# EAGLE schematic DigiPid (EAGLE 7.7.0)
DESIGNER: A. Stummer; GROUP: J. Thywissen Labs; RELEASE_DATE: 2016 Sept; REV: A; TITLE: DigiPid - Digital PID

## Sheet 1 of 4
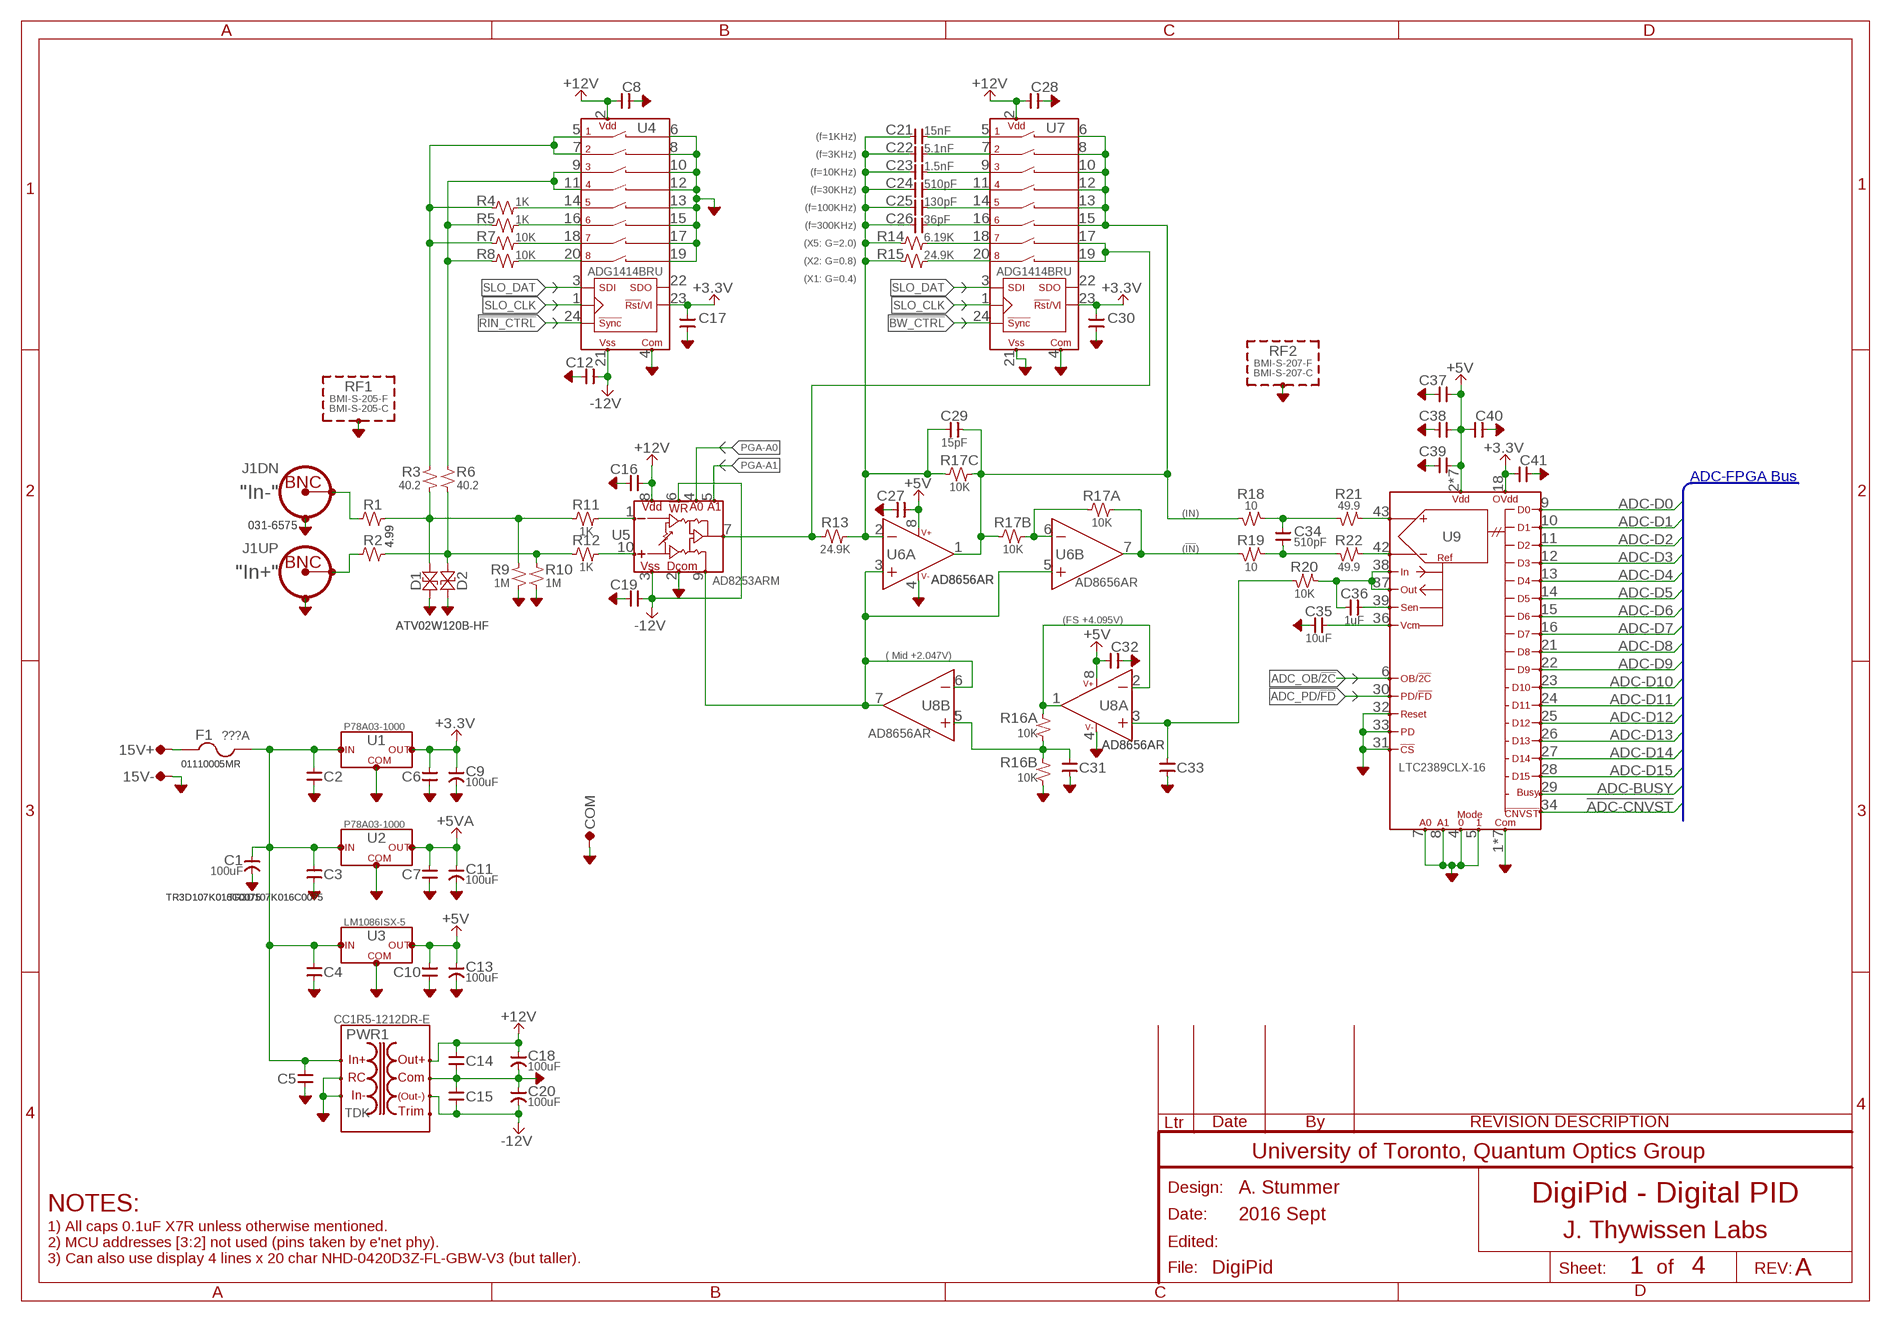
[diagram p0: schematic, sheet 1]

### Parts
15V+  TP-1.5MM  [TP,1.5MM]
15V-  TP-1.5MM  [TP,1.5MM]
C1  100uF  CAP-POL--EIA7343  [7343]
C2  0.1uF  CAP-H-0805  [2012(0805)]
C3  0.1uF  CAP-H-0805  [2012(0805)]
C4  0.1uF  CAP-H-0805  [2012(0805)]
C5  0.1uF  CAP-H-0805  [2012(0805)]
C6  0.1uF  CAP-H-0805  [2012(0805)]
C7  0.1uF  CAP-H-0805  [2012(0805)]
C8  0.1uF  CAP-H-0805  [2012(0805)]
C9  100uF  CAP-POL--EIA7343  [7343]
C10  0.1uF  CAP-H-0805  [2012(0805)]
C11  100uF  CAP-POL--EIA7343  [7343]
C12  0.1uF  CAP-H-0805  [2012(0805)]
C13  100uF  CAP-POL--EIA7343  [7343]
C14  0.1uF  CAP-H-0805  [2012(0805)]
C15  0.1uF  CAP-H-0805  [2012(0805)]
C16  0.1uF  CAP-H-0805  [2012(0805)]
C17  0.1uF  CAP-V-0805  [2012(0805)]
C18  100uF  CAP-POL--EIA7343  [7343]
C19  0.1uF  CAP-H-0805  [2012(0805)]
C20  100uF  CAP-POL--EIA7343  [7343]
C21  15nF  CAP-H-0805  [2012(0805)]
C22  5.1nF  CAP-H-0805  [2012(0805)]
C23  1.5nF  CAP-H-0805  [2012(0805)]
C24  510pF  CAP-H-0805  [2012(0805)]
C25  130pF  CAP-H-0805  [2012(0805)]
C26  36pF  CAP-H-0805  [2012(0805)]
C27  0.1uF  CAP-H-0805  [2012(0805)]
C28  0.1uF  CAP-H-0805  [2012(0805)]
C29  15pF  CAP-H-0805  [2012(0805)]
C30  0.1uF  CAP-V-0805  [2012(0805)]
C31  0.1uF  CAP-H-0805  [2012(0805)]
C32  0.1uF  CAP-H-0805  [2012(0805)]
C33  0.1uF  CAP-H-0805  [2012(0805)]
C34  510pF  CAP-V-0805  [2012(0805)]
C35  10uF  CAP-H-0805  [2012(0805)]
C36  1uF  CAP-H-0805  [2012(0805)]
C37  0.1uF  CAP-H-0805  [2012(0805)]
C38  0.1uF  CAP-H-0805  [2012(0805)]
C39  0.1uF  CAP-H-0805  [2012(0805)]
C40  0.1uF  CAP-H-0805  [2012(0805)]
C41  0.1uF  CAP-H-0805  [2012(0805)]
COM  TP-1MM  [TP-0.042C]
D1  ATV02W120B-HF  TVS,BIPOLAR-SOD123  [SOD123]
D2  ATV02W120B-HF  TVS,BIPOLAR-SOD123  [SOD123]
F1  ???A  FUSE-5X20-4  [FUSE]
J1  031-6575  CONN:BNC,DUAL-BOMAR_364A  [CONN:BNC,DUAL(BOMAR)]
PWR1  CC1R5-1212DR-E  DC-DC:CCP-__-E(TDK1.5-25W)-CC1R5-R-E  [DC-DC:CC1R5-XXXXX-R-E(TDK/LAMBDA)]
R1  4.99  R-H-0805  [2012(0805)]
R2  4.99  R-H-0805  [2012(0805)]
R3  40.2  R-V-0805  [2012(0805)]
R4  1K  R-H-0805  [2012(0805)]
R5  1K  R-H-0805  [2012(0805)]
R6  40.2  R-V-0805  [2012(0805)]
R7  10K  R-H-0805  [2012(0805)]
R8  10K  R-H-0805  [2012(0805)]
R9  1M  R-V-0805  [2012(0805)]
R10  1M  R-V-0805  [2012(0805)]
R11  1K  R-H-0805  [2012(0805)]
R12  1K  R-H-0805  [2012(0805)]
R13  24.9K  R-H-0805  [2012(0805)]
R14  6.19K  R-H-0805  [2012(0805)]
R15  24.9K  R-H-0805  [2012(0805)]
R16  10K  R-4PAK-0603  [PANASONIC_EXB-V8V(QUAD-R-PACK)]
R17  10K  R-4PAK-0603  [PANASONIC_EXB-V8V(QUAD-R-PACK)]
R18  10  R-H-0805  [2012(0805)]
R19  10  R-H-0805  [2012(0805)]
R20  10K  R-H-0805  [2012(0805)]
R21  49.9  R-H-0805  [2012(0805)]
R22  49.9  R-H-0805  [2012(0805)]
RF1  BMI-S-205-F  RF-SHIELD-38X25MM(BMI-S-205-F)  [RF-SHIELD,38X25MM(BMI-S-205-F)]
RF2  BMI-S-207-F  RF-SHIELD-44X44MM(BMI-S-207-F)  [RF-SHIELD,44X44MM(BMI-S-207-F)]
U1  P78A03-1000  REGULATOR:3PIN-SMPS(V-OR-H)  [TO220-SMPS]
U2  P78A03-1000  REGULATOR:3PIN-SMPS(V-OR-H)  [TO220-SMPS]
U3  LM1086ISX-5  REGULATOR:3PIN-TO263  [TO263]
U4  ADG1414BRU  SWITCH,8PST-SERIAL-TSSOP24  [TSSOP-24]
U5  AD8253ARM  ANALOG,INT-AMP-PROG#1-MSOP10  [MSOP10]
U6  AD8656AR  OPAMP:AD8___(DUAL)-SOIC-8  [SOIC-8]
U7  ADG1414BRU  SWITCH,8PST-SERIAL-TSSOP24  [TSSOP-24]
U8  AD8656AR  OPAMP:AD8___(DUAL)-SOIC-8  [SOIC-8]
U9  LTC2389CLX-16  ADC,LTC2389-16-LQFP48  [QFP48]

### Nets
!ADC-CNVST: U9.34(!CNVST) ; also sheet 3
!BW_CTRL: U7.24(!SYNC) ; also sheet 4
!RIN_CTRL: U4.24(!SYNC) ; also sheet 4
+3.3V [Power]: C6.1 C9.+VE(POS) C17.2 C30.2 C41.1 U1.3(OUT) U4.23(!RST!/VL) U7.23(!RST!/VL) U9.18(OVDD) ; also sheet 2,3,4
+5V [Power]: C10.1 C13.+VE(POS) C27.1 C32.1 C37.1 C38.1 C39.1 C40.1 U3.4(OUT) U6.8(PWR:V++) U8.8(PWR:V++) U9.2(VDD) U9.3(VDD) U9.19(VDD) U9.40(VDD) U9.45(VDD) U9.46(VDD) U9.47(VDD) ; also sheet 2,3
+5VA [Power]: C7.1 C11.+VE(POS) U2.3(OUT) ; also sheet 4
+12V [Power]: C8.1 C14.1 C16.1 C18.+VE(POS) C28.1 PWR1.+VOUT(+OUT) U4.2(VDD) U5.8(VDD) U7.2(VDD) ; also sheet 2
-12V [Power]: C12.1 C15.2 C19.1 C20.-VE(NEG) PWR1.-VOUT(-OUT) U4.21(VSS) U5.3(VSS) U5.6(!WR) ; also sheet 2
ADC-BUSY: U9.29(BUSY) ; also sheet 3
ADC-D0: U9.9(D0) ; also sheet 3
ADC-D1: U9.10(D1) ; also sheet 3
ADC-D2: U9.11(D2) ; also sheet 3
ADC-D3: U9.12(D3) ; also sheet 3
ADC-D4: U9.13(D4) ; also sheet 3
ADC-D5: U9.14(D5) ; also sheet 3
ADC-D6: U9.15(D6) ; also sheet 3
ADC-D7: U9.16(D7) ; also sheet 3
ADC-D8: U9.21(D8) ; also sheet 3
ADC-D9: U9.22(D9) ; also sheet 3
ADC-D10: U9.23(D10) ; also sheet 3
ADC-D11: U9.24(D11) ; also sheet 3
ADC-D12: U9.25(D12) ; also sheet 3
ADC-D13: U9.26(D13) ; also sheet 3
ADC-D14: U9.27(D14) ; also sheet 3
ADC-D15: U9.28(D15) ; also sheet 3
ADC_OB/!2C: U9.6(OB!2C) ; also sheet 4
ADC_PD/!FD: U9.30(PD!FD) ; also sheet 4
AGND: 15V-.TP C1.-VE(NEG) C2.2 C3.2 C4.2 C5.2 C6.2 C7.2 C8.2 C9.-VE(NEG) C10.2 C11.-VE(NEG) C12.2 C13.-VE(NEG) C14.2 C15.1 C16.2 C17.1 C18.-VE(NEG) C19.2 C20.+VE(POS) C27.2 C28.2 C30.1 C31.2 C32.2 C33.2 C35.1 C37.2 C38.2 C39.2 C40.2 C41.2 COM.TP D1.C(TOTHER) D2.C(TOTHER) J1.LWR-COM(DN:SHIELD2) J1.UPR-COM(UP:SHIELD2) PWR1.-VIN(-IN) PWR1.COM PWR1.RC R9.1 R10.1 R16.2A RF1.1(SHIELD) RF1.2(SHIELD) RF1.3(SHIELD) RF1.4(SHIELD) RF1.5(SHIELD) RF1.6(SHIELD) RF1.7(SHIELD) RF1.8(SHIELD) RF1.9(SHIELD) RF1.10(SHIELD) RF1.11(SHIELD) RF1.12(SHIELD) RF1.13(SHIELD) RF1.14(SHIELD) RF1.15(SHIELD) RF1.16(SHIELD) RF1.17(SHIELD) RF1.18(SHIELD) RF1.19(SHIELD) RF1.20(SHIELD) RF1.21(SHIELD) RF1.22(SHIELD) RF1.23(SHIELD) RF1.25(SHIELD) RF2.1(SHIELD) RF2.2(SHIELD) RF2.3(SHIELD) RF2.4(SHIELD) RF2.5(SHIELD) RF2.6(SHIELD) RF2.7(SHIELD) RF2.8(SHIELD) RF2.9(SHIELD) RF2.10(SHIELD) RF2.11(SHIELD) RF2.12(SHIELD) RF2.13(SHIELD) RF2.14(SHIELD) RF2.15(SHIELD) RF2.16(SHIELD) RF2.17(SHIELD) RF2.18(SHIELD) RF2.19(SHIELD) RF2.20(SHIELD) RF2.21(SHIELD) RF2.22(SHIELD) RF2.23(SHIELD) RF2.24(SHIELD) RF2.25(SHIELD) RF2.26(SHIELD) RF2.27(SHIELD) RF2.28(SHIELD) RF2.29(SHIELD) RF2.30(SHIELD) RF2.31(SHIELD) RF2.32(SHIELD) U1.2(COM) U2.2(COM) U3.1(COM) U4.4(COM) U4.6(D1) U4.8(D2) U4.10(D3) U4.12(D4) U4.13(D5) U4.15(D6) U4.17(D7) U4.19(D8) U5.2(DGND) U6.4(PWR:V-) U7.4(COM) U7.21(VSS) U8.4(PWR:V-) U9.1(COM) U9.4(MODE0) U9.5(MODE1) U9.7(A0) U9.8(A1) U9.17(COM) U9.20(COM) U9.31(!CS) U9.32(RESET) U9.33(PD) U9.35(COM) U9.41(COM) U9.44(COM) U9.48(COM) ; also sheet 2,3,4
N$1: R3.2 R4.1 R7.1 U4.5(S1) U4.7(S2)
N$2: R5.1 R6.2 R8.1 U4.9(S3) U4.11(S4)
N$3: R13.1 U5.7(OUT) U7.17(D7) U7.19(D8)
N$4: U5.9(REF) U6.3(A:+IN) U6.5(B:+IN) U8.6(B:-IN) U8.7(B:OUT)
N$5: R22.1 U9.42(IN-)
N$6: R21.1 U9.43(IN+)
N$7: C36.2 U9.39(REF-SEN)
N$9: C36.1 R20.1 U9.37(REF-OUT) U9.38(REF-IN)
N$10: C35.2 U9.36(VCM)
N$11: C34.2 R18.1 R21.2
N$12: C34.1 R19.1 R22.2
N$14: R16.1B U8.1(A:OUT) U8.2(A:-IN)
N$17: C21.1 C22.1 C23.1 C24.1 C25.1 C26.1 C29.1 R13.2 R14.1 R15.1 R17.3A U6.2(A:-IN)
N$19: C31.1 R16.1A R16.2B U8.5(B:+IN)
N$30: C33.1 R20.2 U8.3(A:+IN)
N$33: C29.2 R17.2A R17.3B R18.2 U6.1(A:OUT) U7.6(D1) U7.8(D2) U7.10(D3) U7.12(D4) U7.13(D5) U7.15(D6)
N$34: D2.A(ONE) R2.2 R6.1 R10.2 R12.1
N$35: R17.1A R17.2B U6.6(B:-IN)
N$36: R17.1B R19.2 U6.7(B:OUT)
N$37: J1.LWR-CTR(DN:CONDUCTOR) R1.1
N$38: J1.UPR-CTR(UP:CONDUCTOR) R2.1
N$39: D1.A(ONE) R1.2 R3.1 R9.2 R11.1
N$43: R11.2 U5.1(IN-)
N$44: R12.2 U5.10(IN+)
N$45: R15.2 U7.20(S8)
N$46: R14.2 U7.18(S7)
N$47: C26.2 U7.16(S6)
N$48: C25.2 U7.14(S5)
N$49: C24.2 U7.11(S4)
N$52: C23.2 U7.9(S3)
N$53: C22.2 U7.7(S2)
N$58 [Power]: C1.+VE(POS) C2.1 C3.1 C4.1 C5.1 F1.2A F1.2B(2A) PWR1.+VIN(+IN) U1.1(VI) U2.1(VI) U3.3(VI)
N$68: C21.2 U7.5(S1)
N$71: R8.2 U4.20(S8)
N$72: R7.2 U4.18(S7)
N$73: R5.2 U4.16(S6)
N$74: R4.2 U4.14(S5)
N$127 [Power]: 15V+.TP F1.1A F1.1B(1A)
PGA-A0: U5.4(A0) ; also sheet 4
PGA-A1: U5.5(A1) ; also sheet 4
SLO_CLK: U4.1(SCLK) U7.1(SCLK) ; also sheet 2,4
SLO_DAT: U4.3(DIN) U7.3(DIN) ; also sheet 2,4
Unconnected: PWR1.TRM(TRIM) R16.3A R16.3B R16.4A R16.4B R17.4A R17.4B U4.22(SDO) U7.22(SDO)

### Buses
ADC-D[0..15],ADC-BUSY,!ADC-CNVST

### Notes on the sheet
- (f=1KHz)
- (f=3KHz)
- (f=10KHz)
- (f=30KHz)
- (f=100KHz)
- (f=300KHz)
- (X5: G=2.0)
- (X2: G=0.8)
- (X1: G=0.4)
- ADC-FPGA Bus
- "In-"
- (IN)
- (!IN!)
- "In+"
- (FS +4.095V)
- ( Mid +2.047V)
- NOTES:
- 1) All caps 0.1uF X7R unless otherwise mentioned.
  2) MCU addresses [3:2] not used (pins taken by e'net phy).
  3) Can also use display 4 lines x 20 char NHD-0420D3Z-FL-GBW-V3 (but taller).

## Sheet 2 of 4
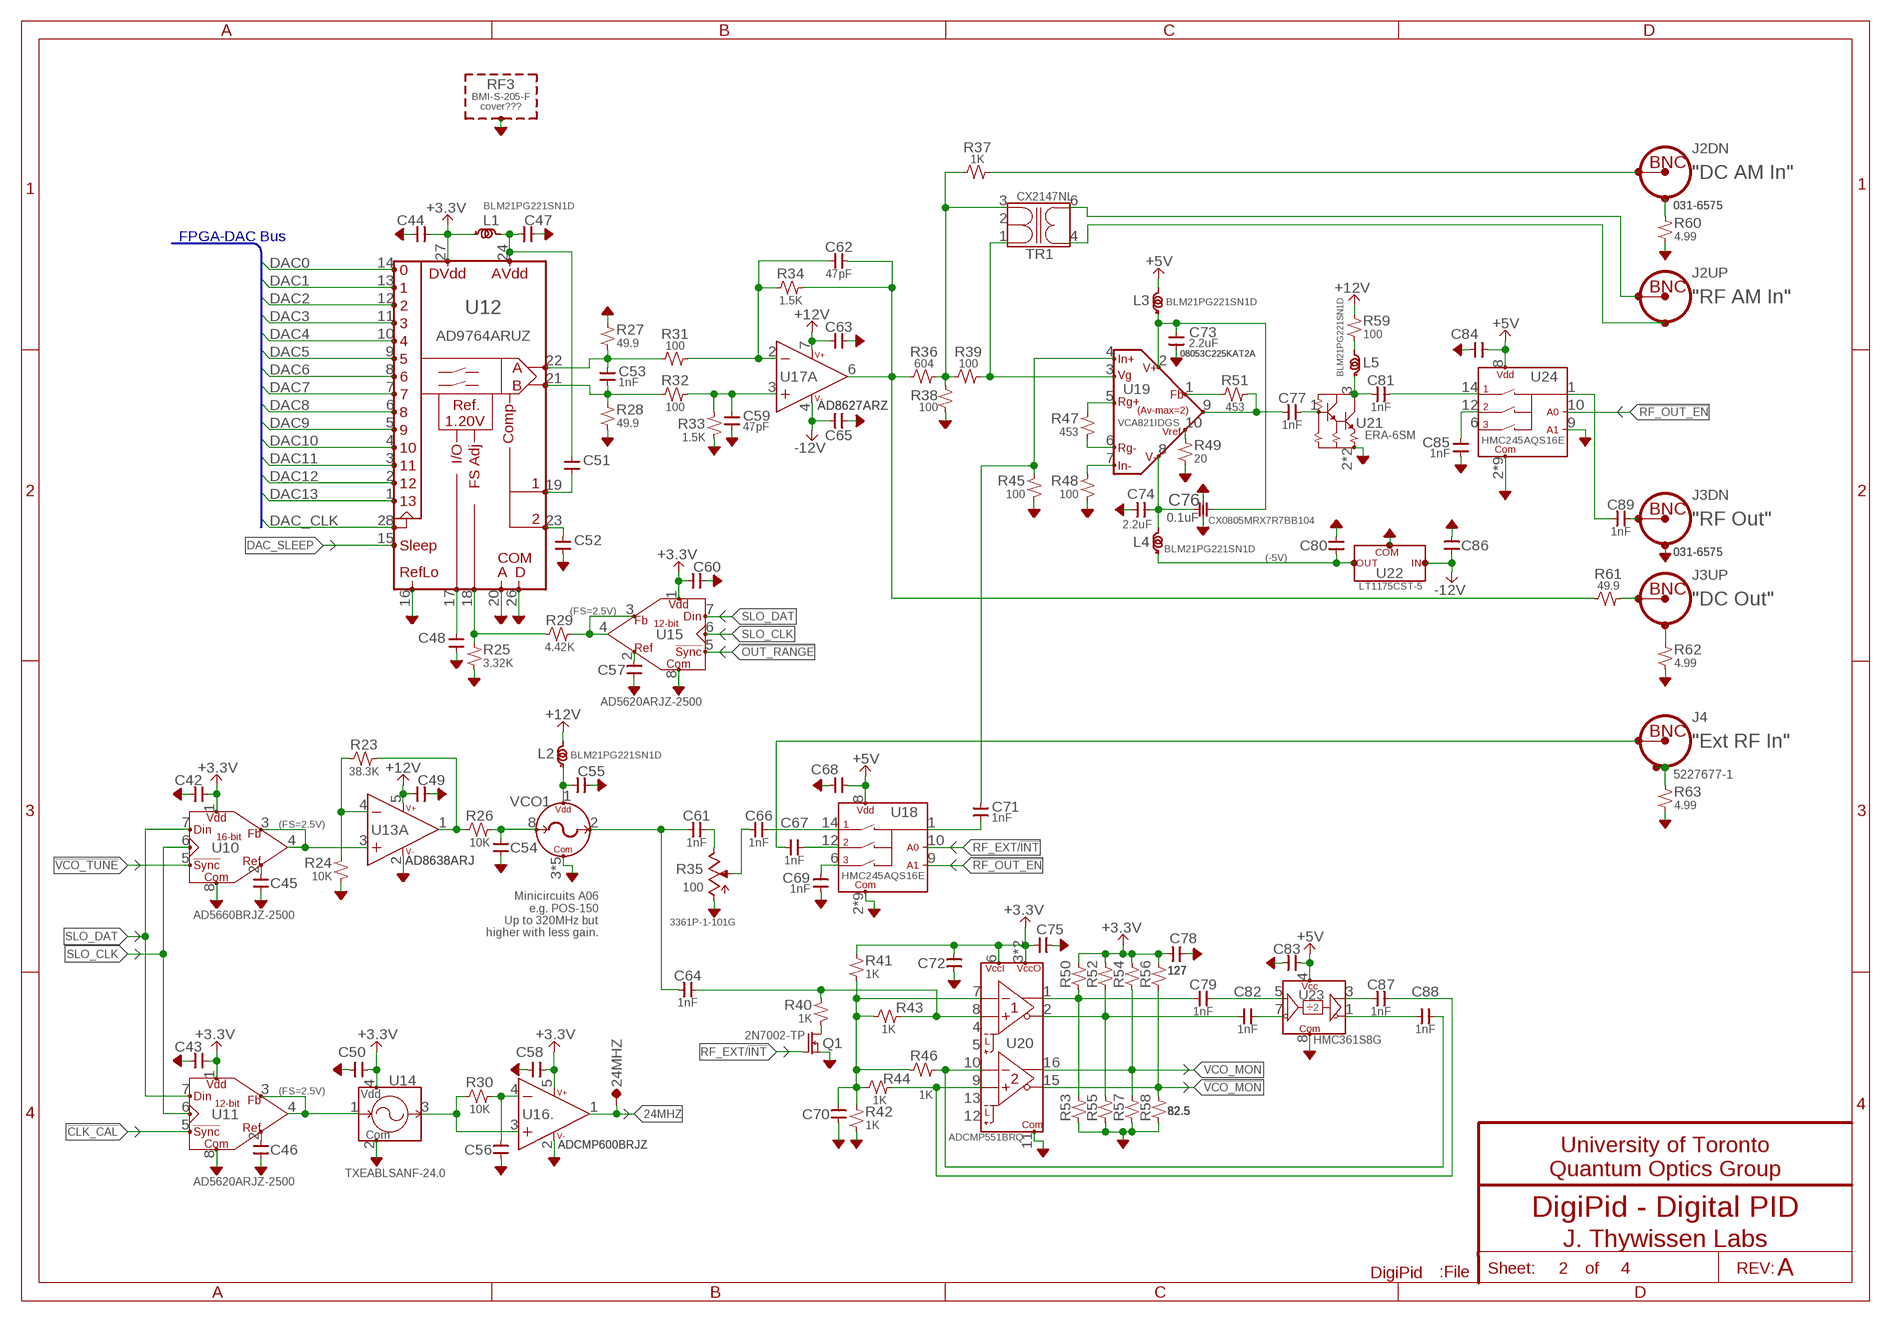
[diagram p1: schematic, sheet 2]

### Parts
24MHZ  TP-0.042B  [TP-0.042B]
C42  0.1uF  CAP-H-0805  [2012(0805)]
C43  0.1uF  CAP-H-0805  [2012(0805)]
C44  0.1uF  CAP-H-0805  [2012(0805)]
C45  0.1uF  CAP-H-0805  [2012(0805)]
C46  0.1uF  CAP-H-0805  [2012(0805)]
C47  0.1uF  CAP-H-0805  [2012(0805)]
C48  0.1uF  CAP-V-0805  [2012(0805)]
C49  0.1uF  CAP-H-0805  [2012(0805)]
C50  0.1uF  CAP-V-0805  [2012(0805)]
C51  0.1uF  CAP-V-0805  [2012(0805)]
C52  0.1uF  CAP-V-0805  [2012(0805)]
C53  1nF  CAP-V-0805  [2012(0805)]
C54  0.1uF  CAP-H-0805  [2012(0805)]
C55  0.1uF  CAP-H-0805  [2012(0805)]
C56  0.1uF  CAP-H-0805  [2012(0805)]
C57  0.1uF  CAP-H-0805  [2012(0805)]
C58  0.1uF  CAP-V-0805  [2012(0805)]
C59  47pF  CAP-V-0805  [2012(0805)]
C60  0.1uF  CAP-H-0805  [2012(0805)]
C61  1nF  CAP-H-0805  [2012(0805)]
C62  47pF  CAP-H-0805  [2012(0805)]
C63  0.1uF  CAP-H-0805  [2012(0805)]
C64  1nF  CAP-H-0805  [2012(0805)]
C65  0.1uF  CAP-H-0805  [2012(0805)]
C66  1nF  CAP-H-0805  [2012(0805)]
C67  1nF  CAP-H-0805  [2012(0805)]
C68  0.1uF  CAP-H-0805  [2012(0805)]
C69  1nF  CAP-V-0805  [2012(0805)]
C70  0.1uF  CAP-H-0805  [2012(0805)]
C71  1nF  CAP-V-0805  [2012(0805)]
C72  0.1uF  CAP-H-0805  [2012(0805)]
C73  2.2uF  CAP-H-0805  [2012(0805)]
C74  2.2uF  CAP-H-0805  [2012(0805)]
C75  0.1uF  CAP-V-0805  [2012(0805)]
C76  0.1uF  CAP-X2Y_DUAL-0603  [1608(0603)X2Y_DUAL]
C77  1nF  CAP-H-0805  [2012(0805)]
C78  0.1uF  CAP-V-0805  [2012(0805)]
C79  1nF  CAP-H-0805  [2012(0805)]
C80  0.1uF  CAP-H-0805  [2012(0805)]
C81  1nF  CAP-H-0805  [2012(0805)]
C82  1nF  CAP-H-0805  [2012(0805)]
C83  0.1uF  CAP-H-0805  [2012(0805)]
C84  0.1uF  CAP-H-0805  [2012(0805)]
C85  1nF  CAP-V-0805  [2012(0805)]
C86  0.1uF  CAP-H-0805  [2012(0805)]
C87  1nF  CAP-H-0805  [2012(0805)]
C88  1nF  CAP-H-0805  [2012(0805)]
C89  1nF  CAP-H-0805  [2012(0805)]
J2  031-6575  CONN:BNC,DUAL-BOMAR_364A  [CONN:BNC,DUAL(BOMAR)]
J3  031-6575  CONN:BNC,DUAL-BOMAR_364A  [CONN:BNC,DUAL(BOMAR)]
J4  5227677-1  CONN:BNCTYPE3HORIZ  [CONN:BNC-AMP-TYPE3HORIZ]
L1  BLM21PG221SN1D  INDUCTOR0805  [2012(0805)]
L2  BLM21PG221SN1D  INDUCTOR0805  [2012(0805)]
L3  BLM21PG221SN1D  INDUCTOR0805  [2012(0805)]
L4  BLM21PG221SN1D  INDUCTOR0805  [2012(0805)]
L5  BLM21PG221SN1D  INDUCTOR0805  [2012(0805)]
Q1  2N7002-TP  MOSFET-N-SOT23  [SOT23]
R23  38.3K  R-H-0805  [2012(0805)]
R24  10K  R-V-0805  [2012(0805)]
R25  3.32K  R-V-0805  [2012(0805)]
R26  10K  R-H-0805  [2012(0805)]
R27  49.9  R-V-0805  [2012(0805)]
R28  49.9  R-V-0805  [2012(0805)]
R29  4.42K  R-H-0805  [2012(0805)]
R30  10K  R-H-0805  [2012(0805)]
R31  100  R-H-0805  [2012(0805)]
R32  100  R-H-0805  [2012(0805)]
R33  1.5K  R-V-0805  [2012(0805)]
R34  1.5K  R-H-0805  [2012(0805)]
R35  100  POT-BOURNS_3361P  [BOURNS_3361P]
R36  604  R-H-0805  [2012(0805)]
R37  1K  R-H-0805  [2012(0805)]
R38  100  R-V-0805  [2012(0805)]
R39  100  R-H-0805  [2012(0805)]
R40  1K  R-V-0805  [2012(0805)]
R41  1K  R-V-0805  [2012(0805)]
R42  1K  R-V-0805  [2012(0805)]
R43  1K  R-H-0805  [2012(0805)]
R44  1K  R-H-0805  [2012(0805)]
R45  100  R-V-0805  [2012(0805)]
R46  1K  R-H-0805  [2012(0805)]
R47  453  R-V-0805  [2012(0805)]
R48  100  R-V-0805  [2012(0805)]
R49  20  R-V-0805  [2012(0805)]
R50  127  R-V-0805  [2012(0805)]
R51  453  R-H-0805  [2012(0805)]
R52  127  R-V-0805  [2012(0805)]
R53  82.5  R-V-0805  [2012(0805)]
R54  127  R-V-0805  [2012(0805)]
R55  82.5  R-V-0805  [2012(0805)]
R56  127  R-V-0805  [2012(0805)]
R57  82.5  R-V-0805  [2012(0805)]
R58  82.5  R-V-0805  [2012(0805)]
R59  100  R-V-0805  [2012(0805)]
R60  4.99  R-V-0805  [2012(0805)]
R61  49.9  R-H-0805  [2012(0805)]
R62  4.99  R-V-0805  [2012(0805)]
R63  4.99  R-V-0805  [2012(0805)]
RF3  BMI-S-205-F  RF-SHIELD-38X25MM(BMI-S-205-F)  [RF-SHIELD,38X25MM(BMI-S-205-F)]
TR1  CX2147NL  TRANSFORMER,5WIRE-PULSE_CX2  [TRANSFORMER,PULSE_CX2___]
U10  AD5660BRJZ-2500  DAC,SERIAL,FDBK-SOT23-8  [SOT23-8]
U11  AD5620ARJZ-2500  DAC,SERIAL,FDBK-SOT23-8  [SOT23-8]
U12  AD9764ARUZ  DAC,AD97X4(14-BIT,125MSPS,PAR)-TSSOP28  [TSSOP-28]
U13  AD8638ARJ  OPAMP-SOT23-5  [SOT23-5]
U14  TXEABLSANF-24.0  OSCILLATOR:CX750(CITIZEN)-TAINTIEN_TW_TX  [OSCILLATOR,TAITIEN_TW_TX]
U15  AD5620ARJZ-2500  DAC,SERIAL,FDBK-SOT23-8  [SOT23-8]
U16  ADCMP600BRJZ  COMPARATOR,SINGLE,SINGLE_SUPPY-SOT23-5(ALT)  [SOT23-5]
U17  AD8627ARZ  OPAMP-SO8  [SOIC-8]
U18  HMC245AQS16E  SWITCH,SP3T,PAR-QSOP16  [QSOP-16(RQ-16)]
U19  VCA821IDGS  LINEAR,VGA,#2-MSOP10  [MSOP10]
U20  ADCMP551BRQ  COMPARATOR,ADCMP551(DUAL,500PS,LVPECL)-QSOP16  [QSOP-16(RQ-16)]
U21  ERA-6SM  RF,AMP#1-MINIC_WW107  [MINICIRCUITS_WW107]
U22  LT1175CST-5  REGULATOR:NEG-3-TERM-SOT223  [SOT223]
U23  HMC361S8G  RF,DIVIDE_BY_N-SOIC8(PAD)  [SOIC8(E-PAD)]
U24  HMC245AQS16E  SWITCH,SP3T,PAR-QSOP16  [QSOP-16(RQ-16)]
VCO1  Minicircuits A06  RF,VCO#1-MINICIRCUITS_A06  [MINICIRCUITS_A06]

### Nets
24MHZ: 24MHZ.TP U16.1(.:OUT) ; also sheet 3,4
!CLK_CAL: U11.5(!SYNC) ; also sheet 4
!OUT_RANGE: U15.5(!SYNC) ; also sheet 4
!RF_OUT_EN: U18.9(A1) U24.10(A0) ; also sheet 3
!VCO_MON: R56.1 R58.2 U20.15(Q-2) ; also sheet 3
!VCO_TUNE: U10.5(!SYNC) ; also sheet 4
+3.3V [Power]: C42.1 C43.1 C44.1 C50.2 C58.2 C60.1 C72.1 C75.2 C78.2 L1.1(A) R41.2 R50.2 R52.2 R54.2 R56.2 U10.1(VDD) U11.1(VDD) U12.27(DVDD) U14.4(VDD) U15.1(VDD) U16.5(V++) U20.3(VCCO) U20.6(VCCI) U20.14(VCCO) ; also sheet 1,3,4
+5V [Power]: C68.2 C83.2 C84.2 L3.2(B) U18.8(VDD) U23.4(VCC) U24.8(VDD) ; also sheet 1,3
+12V [Power]: C49.1 C63.1 L2.2(B) R59.2 U13.5(B:V++) U17.7(B:V++) ; also sheet 1
-12V [Power]: C65.1 C86.2 U17.4(B:V-) U22.2(VI) U22.4(VI) ; also sheet 1
AGND: C42.2 C43.2 C44.2 C45.2 C46.2 C47.2 C48.1 C49.2 C50.1 C52.1 C54.2 C55.2 C56.2 C57.2 C58.1 C59.1 C60.2 C63.2 C65.2 C68.1 C69.1 C70.2 C72.2 C73.2 C74.2 C75.1 C76.COM1 C76.COM2 C78.1 C80.1 C83.1 C84.1 C85.1 C86.1 J3.LWR-COM(DN:SHIELD2) Q1.2(S) R24.1 R25.1 R27.2 R28.1 R33.1 R35.CCW R38.1 R42.1 R45.1 R48.1 R49.1 R53.1 R55.1 R57.1 R58.1 R60.1 R62.1 R63.1 RF3.1(SHIELD) RF3.2(SHIELD) RF3.3(SHIELD) RF3.4(SHIELD) RF3.5(SHIELD) RF3.6(SHIELD) RF3.7(SHIELD) RF3.8(SHIELD) RF3.9(SHIELD) RF3.10(SHIELD) RF3.11(SHIELD) RF3.12(SHIELD) RF3.13(SHIELD) RF3.14(SHIELD) RF3.15(SHIELD) RF3.16(SHIELD) RF3.17(SHIELD) RF3.18(SHIELD) RF3.19(SHIELD) RF3.20(SHIELD) RF3.21(SHIELD) RF3.22(SHIELD) RF3.23(SHIELD) RF3.25(SHIELD) U10.8(COM) U11.8(COM) U12.16(REFLO) U12.20(ACOM) U12.26(DCOM) U13.2(B:V-) U14.2(COM) U15.8(COM) U16.2(V-) U18.2(COM) U18.3(COM) U18.4(COM) U18.5(COM) U18.7(COM) U18.11(COM) U18.13(COM) U18.15(COM) U18.16(COM) U20.11(COM) U21.2(COM) U21.4(COM) U22.3(COM) U23.8(COM) U24.2(COM) U24.3(COM) U24.4(COM) U24.5(COM) U24.7(COM) U24.9(A1) U24.11(COM) U24.13(COM) U24.15(COM) U24.16(COM) VCO1.3(COM) VCO1.4(COM) VCO1.5(COM) VCO1.6(COM) VCO1.7(COM) ; also sheet 1,3,4
DAC0: U12.14 ; also sheet 3
DAC1: U12.13 ; also sheet 3
DAC2: U12.12 ; also sheet 3
DAC3: U12.11 ; also sheet 3
DAC4: U12.10 ; also sheet 3
DAC5: U12.9 ; also sheet 3
DAC6: U12.8 ; also sheet 3
DAC7: U12.7 ; also sheet 3
DAC8: U12.6 ; also sheet 3
DAC9: U12.5 ; also sheet 3
DAC10: U12.4 ; also sheet 3
DAC11: U12.3 ; also sheet 3
DAC12: U12.2 ; also sheet 3
DAC13: U12.1 ; also sheet 3
DAC_CLK: U12.28(CLK) ; also sheet 3
DAC_SLEEP: U12.15(SLEEP) ; also sheet 4
N$18: R51.1 U19.1(FB)
N$20: R25.2 R29.1 U12.18(FSADJ)
N$21: C46.1 U11.2(REFOUT)
N$22: C48.2 U12.17(REF)
N$23: C52.2 U12.23(COMP2)
N$24: C53.2 R27.1 R31.1 U12.22(IOUTA)
N$25: C53.1 R28.2 R32.1 U12.21(IOUTB)
N$26: C80.2 L4.1(A) U22.1(OUT)
N$27: C62.1 R31.2 R34.1 U17.2(A:-IN)
N$28: C59.2 R32.2 R33.2 U17.3(A:+IN)
N$29: J3.UPR-CTR(UP:CONDUCTOR) R61.2
N$32: C47.1 C51.2 L1.2(B) U12.24(AVDD)
N$41: R47.2 U19.5(RG+)
N$69: C57.1 U15.2(REFOUT)
N$70: R29.2 U15.3(FB) U15.4(OUT)
N$75: U11.3(FB) U11.4(OUT) U14.1(EN)
N$76: C77.1 U21.1(IN)
N$77: R48.2 U19.7(IN-)
N$78: C61.1 R35.CW
N$79: R47.1 U19.6(RG-)
N$80: R49.2 U19.10(VREF)
N$81: R36.2 R37.1 R38.2 R39.1 TR1.3(S-)
N$82: C71.1 U18.1(D)
N$83: C66.2 R35.W
N$84 [Microstrip_50]: C67.2 J4.CONDUCTOR
N$85: C69.2 U18.6(S3)
N$86: R23.1 R24.2 U13.4(A:-IN)
N$87: C66.1 U18.14(S1)
N$88: C61.2 C64.2 VCO1.2(OUT)
N$89: C67.1 U18.12(S2)
N$90: C45.1 U10.2(REFOUT)
N$91: C73.1 C76.2 L3.1(A) U19.2(V+)
N$92: U10.3(FB) U10.4(OUT) U13.3(A:+IN)
N$93 [Microstrip_50]: C71.2 R45.2 U19.4(IN+)
N$94: C55.1 L2.1(A) VCO1.1(VDD)
N$96: C85.2 U24.12(S2)
N$97: C81.1 U24.14(S1)
N$98 [Microstrip_50]: C89.2 U24.1(D)
N$99: R39.2 TR1.1(S+) U19.3(VG)
N$100 [Microstrip_50]: C89.1 J3.LWR-CTR(DN:CONDUCTOR)
N$101: J2.UPR-CTR(UP:CONDUCTOR) TR1.6(P-)
N$103: C54.1 R26.2 VCO1.8(VTUNE)
N$104: R23.2 R26.1 U13.1(A:OUT)
N$105: C62.2 R34.2 R36.1 R61.1 U17.6(A:OUT)
N$106: C56.1 R30.2 U16.4(.:-IN)
N$108: C77.2 R51.2 U19.9(OUT)
N$109: L5.2(B) R59.1
N$110 [Microstrip_50]: C81.2 L5.1(A) U21.3(OUT)
N$123: C74.1 C76.1 L4.2(B) U19.8(V-)
N$140: J3.UPR-COM(UP:SHIELD2) R62.2
N$144: R30.1 U14.3(Q) U16.3(.:+IN)
N$147: J2.LWR-CTR(DN:CONDUCTOR) R37.2
N$172: C88.1 R46.2 U20.10(IN-2)
N$173: C70.1 R41.1 R42.2 R43.1 R44.1 R46.1 U20.7(IN-1)
N$175: J4.SHIELD1 J4.SHIELD2 R63.2
N$194: J2.LWR-COM(DN:SHIELD2) R60.2
N$199: C51.1 U12.19(COMP1)
N$202: C64.1 R40.2 R43.2 U20.8(IN+1)
N$204: C79.2 R50.1 R53.2 U20.1(Q+1)
N$205: C82.2 R52.1 R55.2 U20.2(Q-1)
N$206: C88.2 U23.1(!Q)
N$208: C79.1 U23.5(IN)
N$209: C82.1 U23.7(!IN)
N$210: C87.1 R44.2 U20.9(IN+2)
N$211: J2.UPR-COM(UP:SHIELD2) TR1.4(P+)
N$212: Q1.3(D) R40.1
N$213: C87.2 U23.3(Q)
RF_EXT/!INT: Q1.1(G) U18.10(A0) ; also sheet 4
SLO_CLK: U10.6(SCLK) U11.6(SCLK) U15.6(SCLK) ; also sheet 1,4
SLO_DAT: U10.7(SDI) U11.7(SDI) U15.7(SDI) ; also sheet 1,4
VCO_MON: R54.1 R57.2 U20.16(Q+2) ; also sheet 3
Unconnected: TR1.2(SCT) U20.4(LA+1) U20.5(LA-1) U20.12(LA-2) U20.13(LA+2) U24.6(S3)

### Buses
DAC[0..13],DAC_CLK

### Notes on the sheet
- "DC AM In"
- FPGA-DAC Bus
- "RF AM In"
- (Av-max=2)
- "RF Out"
- (-5V)
- "DC Out"
- (FS=2.5V)
- 12-bit
- "Ext RF In"
- (FS=2.5V)
- 16-bit
- e.g. POS-150
  Up to 320MHz but
  higher with less gain.
- (FS=2.5V)
- 12-bit

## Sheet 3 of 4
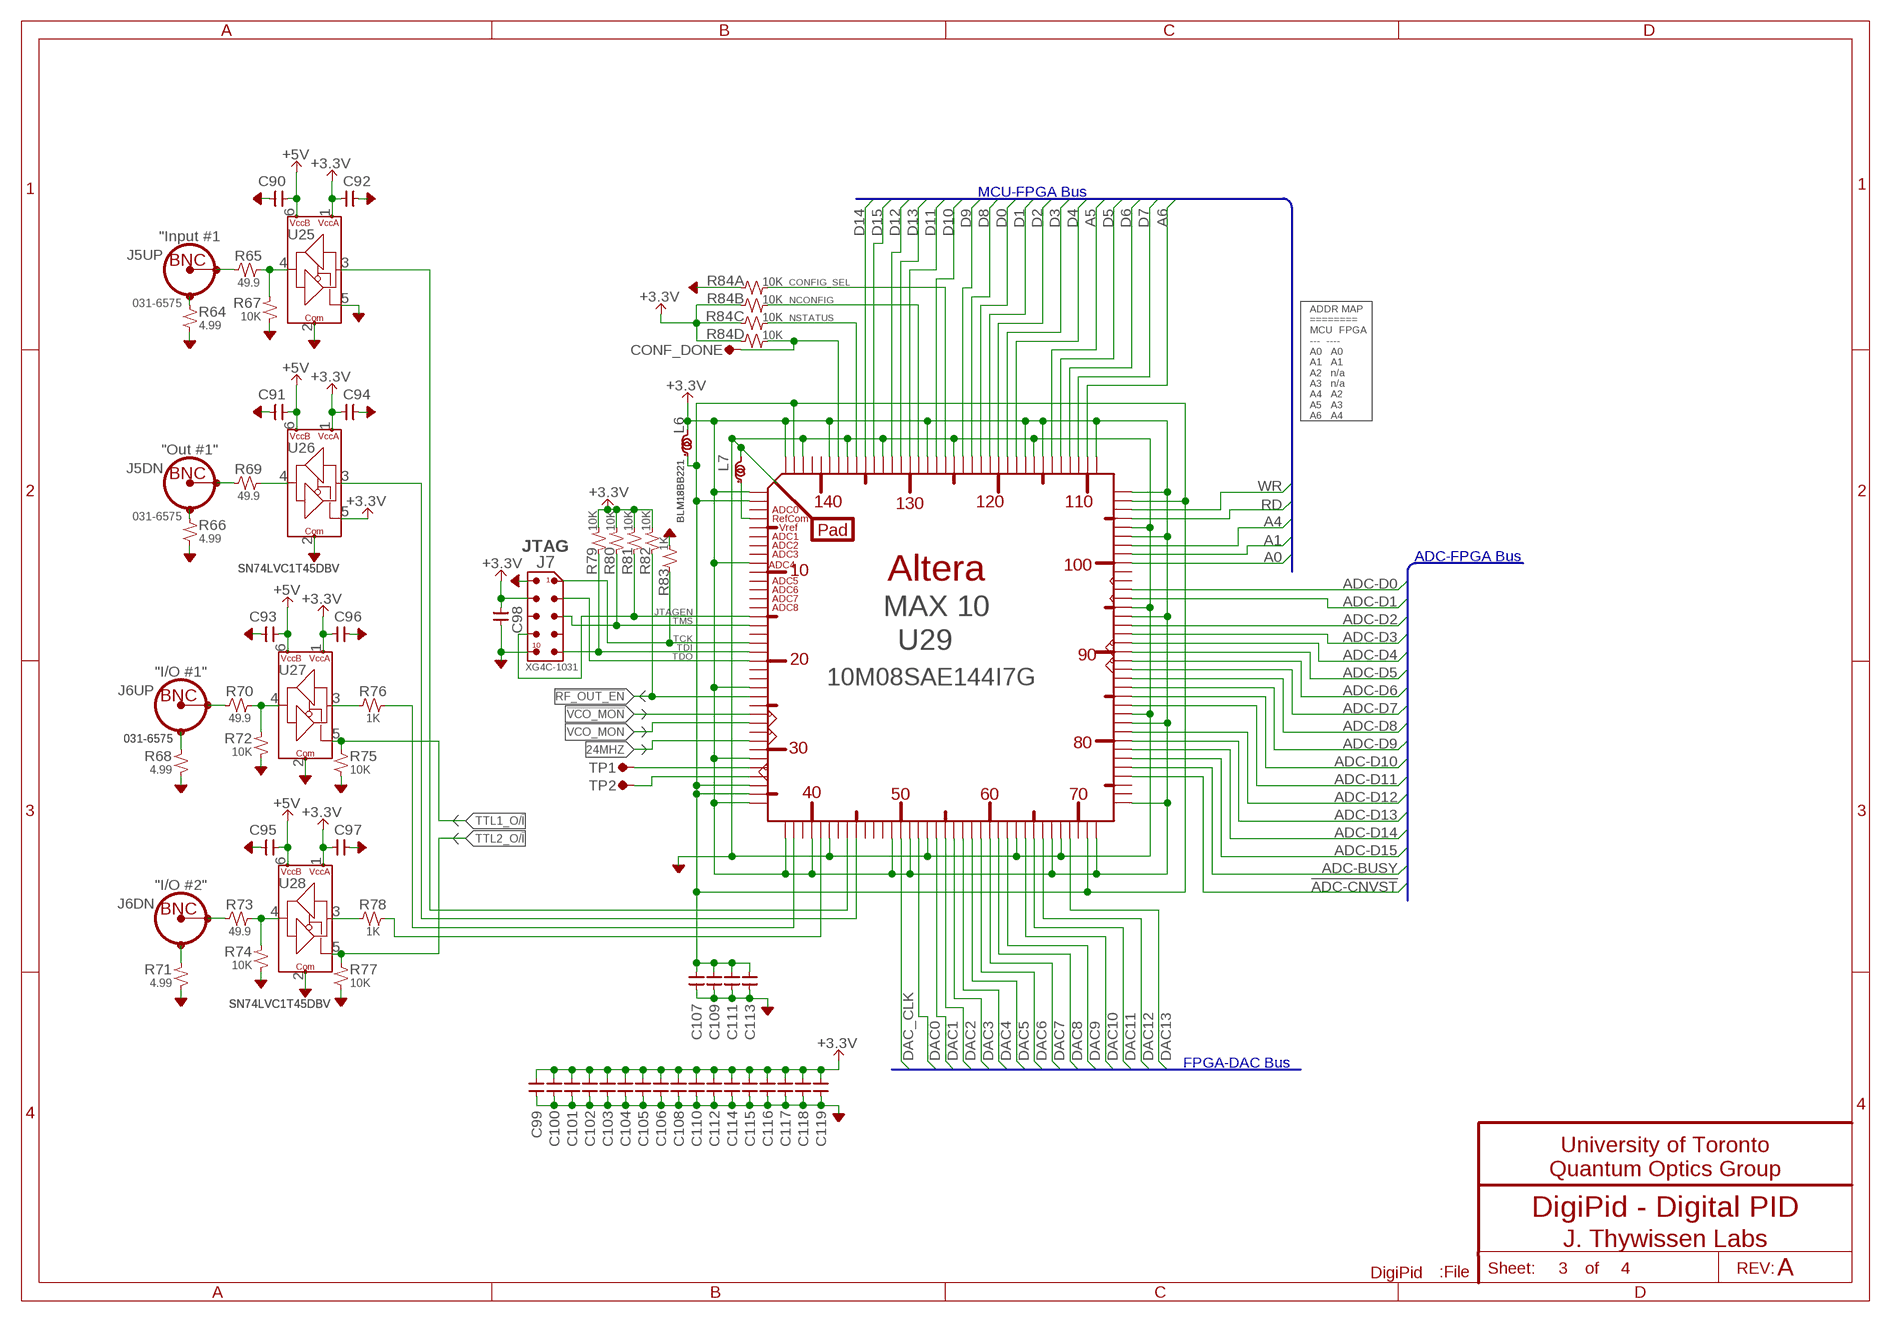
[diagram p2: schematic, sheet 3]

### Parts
C90  0.1uF  CAP-V-0805  [2012(0805)]
C91  0.1uF  CAP-V-0805  [2012(0805)]
C92  0.1uF  CAP-V-0805  [2012(0805)]
C93  0.1uF  CAP-V-0805  [2012(0805)]
C94  0.1uF  CAP-V-0805  [2012(0805)]
C95  0.1uF  CAP-V-0805  [2012(0805)]
C96  0.1uF  CAP-V-0805  [2012(0805)]
C97  0.1uF  CAP-V-0805  [2012(0805)]
C98  0.1uF  CAP-V-0805  [2012(0805)]
C99  0.1uF  CAP-V-0603  [1608(0603)]
C100  0.1uF  CAP-V-0603  [1608(0603)]
C101  0.1uF  CAP-V-0603  [1608(0603)]
C102  0.1uF  CAP-V-0603  [1608(0603)]
C103  0.1uF  CAP-V-0603  [1608(0603)]
C104  0.1uF  CAP-V-0603  [1608(0603)]
C105  0.1uF  CAP-V-0603  [1608(0603)]
C106  0.1uF  CAP-V-0603  [1608(0603)]
C107  0.1uF  CAP-V-0603  [1608(0603)]
C108  0.1uF  CAP-V-0603  [1608(0603)]
C109  0.1uF  CAP-V-0603  [1608(0603)]
C110  0.1uF  CAP-V-0603  [1608(0603)]
C111  0.1uF  CAP-V-0603  [1608(0603)]
C112  0.1uF  CAP-V-0603  [1608(0603)]
C113  0.1uF  CAP-V-0603  [1608(0603)]
C114  0.1uF  CAP-V-0603  [1608(0603)]
C115  0.1uF  CAP-V-0603  [1608(0603)]
C116  0.1uF  CAP-V-0603  [1608(0603)]
C117  0.1uF  CAP-V-0603  [1608(0603)]
C118  0.1uF  CAP-V-0603  [1608(0603)]
C119  0.1uF  CAP-V-0603  [1608(0603)]
CONF_DONE  TP-1MM  [TP-0.042C]
J5  031-6575  CONN:BNC,DUAL-BOMAR_364A  [CONN:BNC,DUAL(BOMAR)]
J6  031-6575  CONN:BNC,DUAL-BOMAR_364A  [CONN:BNC,DUAL(BOMAR)]
J7  XG4C-1031  CONN:2X5-BLASTER-THROUGH  [CONN:2X5-BLASTER]
L6  BLM18BB221  INDUCTOR-0603  [1608(0603)]
L7  BLM18BB221  INDUCTOR-0603  [1608(0603)]
R64  4.99  R-V-0805  [2012(0805)]
R65  49.9  R-H-0805  [2012(0805)]
R66  4.99  R-V-0805  [2012(0805)]
R67  10K  R-V-0805  [2012(0805)]
R68  4.99  R-V-0805  [2012(0805)]
R69  49.9  R-H-0805  [2012(0805)]
R70  49.9  R-H-0805  [2012(0805)]
R71  4.99  R-V-0805  [2012(0805)]
R72  10K  R-V-0805  [2012(0805)]
R73  49.9  R-H-0805  [2012(0805)]
R74  10K  R-V-0805  [2012(0805)]
R75  10K  R-V-0805  [2012(0805)]
R76  1K  R-H-0805  [2012(0805)]
R77  10K  R-V-0805  [2012(0805)]
R78  1K  R-H-0805  [2012(0805)]
R79  10K  R-V-0805  [2012(0805)]
R80  10K  R-V-0805  [2012(0805)]
R81  10K  R-V-0805  [2012(0805)]
R82  10K  R-V-0805  [2012(0805)]
R83  1K  R-V-0805  [2012(0805)]
R84  10K  R-4PAK-0603  [PANASONIC_EXB-V8V(QUAD-R-PACK)]
TP1  TP-1MM  [TP-0.042C]
TP2  TP-1MM  [TP-0.042C]
U25  SN74LVC1T45DBV  LOGIC,BUFFER,BIDIR,1-BIT-SOT23-6  [SOT23-6]
U26  SN74LVC1T45DBV  LOGIC,BUFFER,BIDIR,1-BIT-SOT23-6  [SOT23-6]
U27  SN74LVC1T45DBV  LOGIC,BUFFER,BIDIR,1-BIT-SOT23-6  [SOT23-6]
U28  SN74LVC1T45DBV  LOGIC,BUFFER,BIDIR,1-BIT-SOT23-6  [SOT23-6]
U29  10M08SAE144I7G  FPGA_EP4C_T144(CYCLONE4)EQFP_ONE_VIA  [EQFP144(TQFP_WITH_GROUND_PAD)]

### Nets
24MHZ: U29.29 ; also sheet 2,4
!ADC-CNVST: U29.76 ; also sheet 1
!RF_OUT_EN: R82.1 U29.24 ; also sheet 2
!VCO_MON: U29.26 ; also sheet 2
+3.3V [Power]: C92.2 C94.2 C96.2 C97.2 C98.2 C99.2 C100.2 C101.2 C102.2 C103.2 C104.2 C105.2 C106.2 C108.2 C110.2 C112.2 C114.2 C115.2 C116.2 C117.2 C118.2 C119.2 J7.4 L6.2(B) R79.2 R80.2 R81.2 R82.2 R84.2A R84.3A R84.4A U25.1(VCCA) U26.1(VCCA) U26.5(DIR) U27.1(VCCA) U28.1(VCCA) U29.1 U29.9 U29.23 U29.31 U29.36 U29.37 U29.40 U29.49 U29.51 U29.67 U29.72 U29.73 U29.82 U29.94 U29.103 U29.108 U29.109 U29.115 U29.117 U29.128 U29.139 U29.144 ; also sheet 1,2,4
+3.3VF [Power,0.25mm]: C107.2 C109.2 C111.2 C113.2 L6.1(A) U29.2 U29.34 U29.35 U29.71 U29.107 U29.143
+5V [Power]: C90.2 C91.2 C93.2 C95.2 U25.6(VCCB) U26.6(VCCB) U27.6(VCCB) U28.6(VCCB) ; also sheet 1,2
A0: U29.100 ; also sheet 4
A1: U29.101 ; also sheet 4
A4: U29.102 ; also sheet 4
A5: U29.114 ; also sheet 4
A6: U29.110 ; also sheet 4
ADC-BUSY: U29.77 ; also sheet 1
ADC-D0: U29.97 ; also sheet 1
ADC-D1: U29.96 ; also sheet 1
ADC-D2: U29.93 ; also sheet 1
ADC-D3: U29.92 ; also sheet 1
ADC-D4: U29.91 ; also sheet 1
ADC-D5: U29.90 ; also sheet 1
ADC-D6: U29.89 ; also sheet 1
ADC-D7: U29.88 ; also sheet 1
ADC-D8: U29.87 ; also sheet 1
ADC-D9: U29.86 ; also sheet 1
ADC-D10: U29.85 ; also sheet 1
ADC-D11: U29.84 ; also sheet 1
ADC-D12: U29.81 ; also sheet 1
ADC-D13: U29.80 ; also sheet 1
ADC-D14: U29.79 ; also sheet 1
ADC-D15: U29.78 ; also sheet 1
AGND: C90.1 C91.1 C92.1 C93.1 C94.1 C95.1 C96.1 C97.1 C98.1 C99.1 C100.1 C101.1 C102.1 C103.1 C104.1 C105.1 C106.1 C107.1 C108.1 C109.1 C110.1 C111.1 C112.1 C113.1 C114.1 C115.1 C116.1 C117.1 C118.1 C119.1 J7.2 J7.10 L7.2(B) R64.1 R66.1 R67.1 R68.1 R71.1 R72.1 R74.1 R75.1 R77.1 R83.2 R84.1A U25.2(COM) U25.5(DIR) U26.2(COM) U27.2(COM) U28.2(COM) U29.42 U29.53 U29.63 U29.68 U29.83 U29.95 U29.104 U29.116 U29.125 U29.133 U29.137 U29.142 U29.PAD ; also sheet 1,2,4
CONFIG_SEL: R84.1B U29.126
D0: U29.122 ; also sheet 4
D1: U29.121 ; also sheet 4
D2: U29.120 ; also sheet 4
D3: U29.119 ; also sheet 4
D4: U29.118 ; also sheet 4
D5: U29.113 ; also sheet 4
D6: U29.112 ; also sheet 4
D7: U29.111 ; also sheet 4
D8: U29.123 ; also sheet 4
D9: U29.124 ; also sheet 4
D10: U29.127 ; also sheet 4
D11: U29.130 ; also sheet 4
D12: U29.132 ; also sheet 4
D13: U29.131 ; also sheet 4
D14: U29.135 ; also sheet 4
D15: U29.134 ; also sheet 4
DAC0: U29.52 ; also sheet 2
DAC1: U29.54 ; also sheet 2
DAC2: U29.55 ; also sheet 2
DAC3: U29.56 ; also sheet 2
DAC4: U29.57 ; also sheet 2
DAC5: U29.58 ; also sheet 2
DAC6: U29.59 ; also sheet 2
DAC7: U29.60 ; also sheet 2
DAC8: U29.61 ; also sheet 2
DAC9: U29.62 ; also sheet 2
DAC10: U29.64 ; also sheet 2
DAC11: U29.65 ; also sheet 2
DAC12: U29.66 ; also sheet 2
DAC13: U29.69 ; also sheet 2
DAC_CLK: U29.50 ; also sheet 2
JTAGEN: J7.8 R81.1 U29.15
N$15: L7.1(A) U29.4
N$16: CONF_DONE.TP R84.4B U29.138
N$50: TP1.TP U29.32
N$51: TP2.TP U29.33
N$54: R73.2 R74.2 U28.4(B)
N$55: R70.2 R72.2 U27.4(B)
N$56: J6.LWR-CTR(DN:CONDUCTOR) R73.1
N$57: J6.UPR-CTR(UP:CONDUCTOR) R70.1
N$60: R76.2 U29.38
N$61: R78.2 U29.41
N$62: R69.2 U26.4(B)
N$63: R65.2 R67.2 U25.4(B)
N$64: J5.LWR-CTR(DN:CONDUCTOR) R69.1
N$65: J5.UPR-CTR(UP:CONDUCTOR) R65.1
N$66: U26.3(A) U29.45
N$67: U25.3(A) U29.44
N$201: R78.1 U28.3(A)
N$207: R76.1 U27.3(A)
N$216: J6.LWR-COM(DN:SHIELD2) R71.2
N$217: J6.UPR-COM(UP:SHIELD2) R68.2
N$218: J5.LWR-COM(DN:SHIELD2) R66.2
N$219: J5.UPR-COM(UP:SHIELD2) R64.2
NCONFIG: R84.2B U29.129
NSTATUS: R84.3B U29.136
RD: U29.105 ; also sheet 4
TCK: J7.1 R83.1 U29.18
TDI: J7.9 R79.1 U29.19
TDO: J7.3 U29.20
TMS: J7.5 R80.1 U29.16
TTL1_O/!I!: R75.2 U27.5(DIR) ; also sheet 4
TTL2_O/!I!: R77.2 U28.5(DIR) ; also sheet 4
VCO_MON: U29.27 ; also sheet 2
WR: U29.106 ; also sheet 4
Unconnected: J7.6 J7.7 U29.3 U29.5 U29.6 U29.7 U29.8 U29.10 U29.11 U29.12 U29.13 U29.14 U29.17 U29.21 U29.22 U29.25 U29.28 U29.30 U29.39 U29.43 U29.46 U29.47 U29.48 U29.70 U29.74 U29.75 U29.98 U29.99 U29.140 U29.141

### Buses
DAC[0..13],DAC_CLK
ADC-D[0..15],ADC-BUSY,!ADC-CNVST
D[0..15],A[0..6],RD,WR

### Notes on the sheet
- MCU-FPGA Bus
- "Input #1
- ADDR MAP
  ========
  MCU  FPGA
  ---  ----
  A0   A0
  A1   A1
  A2   n/a
  A3   n/a
  A4   A2
  A5   A3
  A6   A4
- "Out #1"
- ADC0
- RefCom
- Vref
- ADC1
- ADC2
- JTAG | ADC3
- ADC-FPGA Bus
- ADC4
- ADC5
- ADC6
- ADC7
- ADC8
- "I/O #1"
- "I/O #2"
- FPGA-DAC Bus

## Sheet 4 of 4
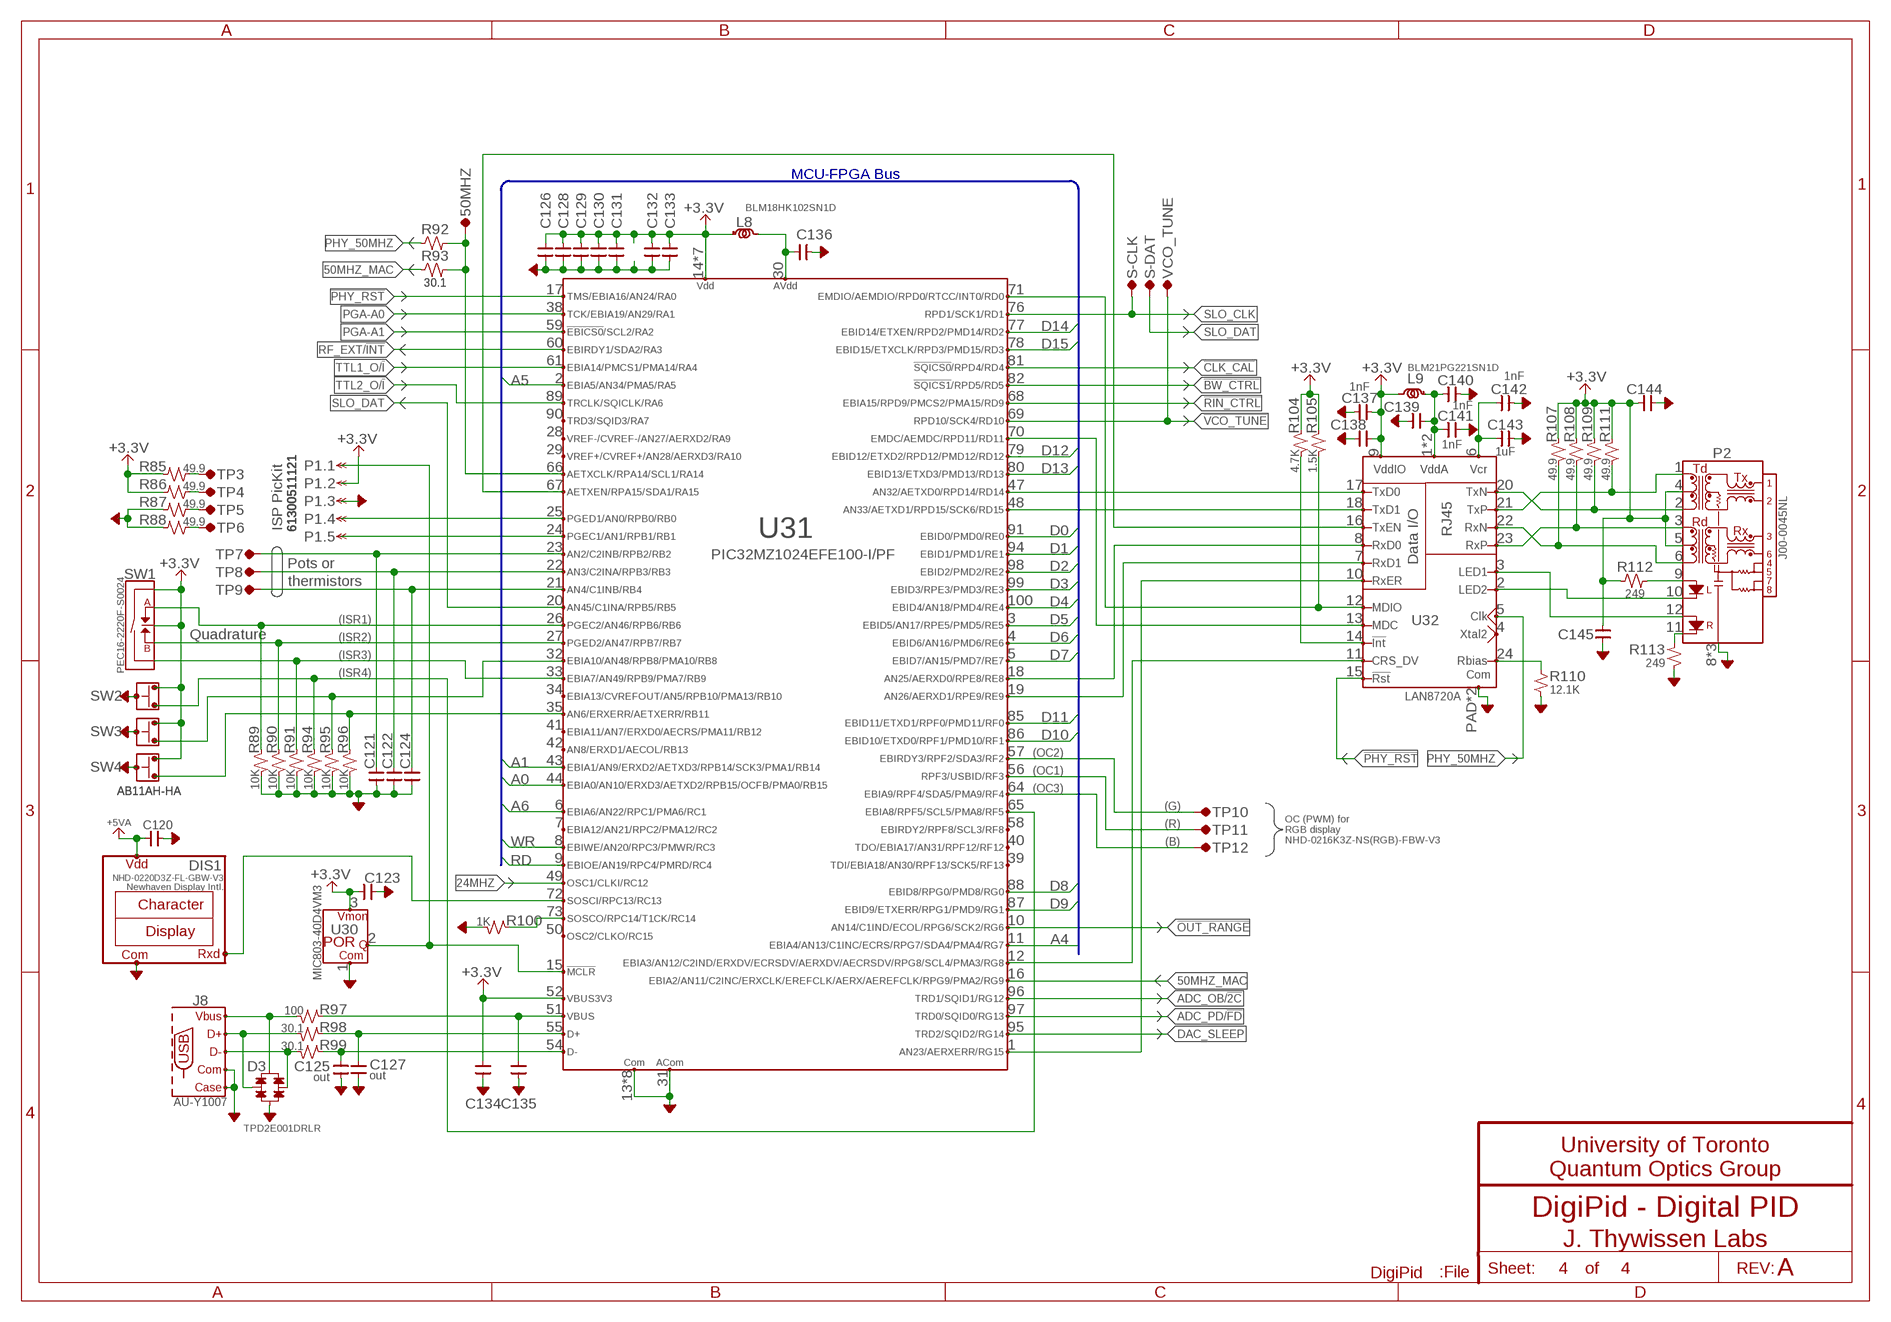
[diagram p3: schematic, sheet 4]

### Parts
50MHZ  TP-0.042B  [TP-0.042B]
C120  0.1uF  CAP-H-0805  [2012(0805)]
C121  0.1uF  CAP-V-0805  [2012(0805)]
C122  0.1uF  CAP-V-0805  [2012(0805)]
C123  0.1uF  CAP-H-0805  [2012(0805)]
C124  0.1uF  CAP-V-0805  [2012(0805)]
C125  out  CAP-V-0805  [2012(0805)]
C126  0.1uF  CAP-V-0805  [2012(0805)]
C127  out  CAP-V-0805  [2012(0805)]
C128  0.1uF  CAP-V-0805  [2012(0805)]
C129  0.1uF  CAP-V-0805  [2012(0805)]
C130  0.1uF  CAP-V-0805  [2012(0805)]
C131  0.1uF  CAP-V-0805  [2012(0805)]
C132  0.1uF  CAP-V-0805  [2012(0805)]
C133  0.1uF  CAP-V-0805  [2012(0805)]
C134  0.1uF  CAP-H-0805  [2012(0805)]
C135  0.1uF  CAP-H-0805  [2012(0805)]
C136  0.1uF  CAP-V-0805  [2012(0805)]
C137  1nF  CAP-H-0805  [2012(0805)]
C138  0.1uF  CAP-H-0805  [2012(0805)]
C139  0.1uF  CAP-H-0805  [2012(0805)]
C140  1nF  CAP-H-0805  [2012(0805)]
C141  1nF  CAP-H-0805  [2012(0805)]
C142  1nF  CAP-H-0805  [2012(0805)]
C143  1uF  CAP-H-0805  [2012(0805)]
C144  0.1uF  CAP-H-0805  [2012(0805)]
C145  0.1uF  CAP-H-0805  [2012(0805)]
D3  TPD2E001DRLR  DIODES,ESD-PROTECTION-SOT553(TI-DRL)  [SOT553]
DIS1  NHD-0220D3Z-FL-GBW-V3  DISPLAY:3WIRE  [DISPLAY:3WIRE]
J8  AU-Y1007  CONN,USB-AUY1007-USB-B  [CONN,USB_AU-Y1007]
L8  BLM18HK102SN1D  INDUCTOR-0603  [1608(0603)]
L9  BLM21PG221SN1D  INDUCTOR0805  [2012(0805)]
P1  61300511121  CONN:1X5-TYPE1-100MIL  [CONN,1X5,100MIL]
P2  J00-0045NL  CONN,RJ45_WITH_MAGNETICS_LEDS#1-PULSE_J00-00  [CONN,RJ45_WITH_MAGNETICS_LEDS#1]
R85  49.9  R-V-0805  [2012(0805)]
R86  49.9  R-V-0805  [2012(0805)]
R87  49.9  R-V-0805  [2012(0805)]
R88  49.9  R-V-0805  [2012(0805)]
R89  10K  R-H-0805  [2012(0805)]
R90  10K  R-H-0805  [2012(0805)]
R91  10K  R-H-0805  [2012(0805)]
R92  30.1  R-H-0805  [2012(0805)]
R93  30.1  R-H-0805  [2012(0805)]
R94  10K  R-H-0805  [2012(0805)]
R95  10K  R-H-0805  [2012(0805)]
R96  10K  R-H-0805  [2012(0805)]
R97  100  R-H-0805  [2012(0805)]
R98  30.1  R-H-0805  [2012(0805)]
R99  30.1  R-H-0805  [2012(0805)]
R100  1K  R-H-0805  [2012(0805)]
R104  4.7K  R-H-0805  [2012(0805)]
R105  1.5K  R-H-0805  [2012(0805)]
R107  49.9  R-H-0805  [2012(0805)]
R108  49.9  R-H-0805  [2012(0805)]
R109  49.9  R-H-0805  [2012(0805)]
R110  12.1K  R-V-0805  [2012(0805)]
R111  49.9  R-H-0805  [2012(0805)]
R112  249  R-H-0805  [2012(0805)]
R113  249  R-V-0805  [2012(0805)]
S-CLK  TP-1MM  [TP-0.042C]
S-DAT  TP-1MM  [TP-0.042C]
SW1  PEC16-2220F-S0024  SWITCH,QUADRATURE+PUSHSWITCH-BOURS_PE16  [SWITCH,QUADRATURE+PUSHSWITCH(BOURNS_PE16)]
SW2  AB11AH-HA  SWITCH,SPST_W-CASE  [SWITCH,SPST,NKK_AB11AH]
SW3  AB11AH-HA  SWITCH,SPST_W-CASE  [SWITCH,SPST,NKK_AB11AH]
SW4  AB11AH-HA  SWITCH,SPST_W-CASE  [SWITCH,SPST,NKK_AB11AH]
TP3  TP-0.042B  [TP-0.042B]
TP4  TP-0.042B  [TP-0.042B]
TP5  TP-0.042B  [TP-0.042B]
TP6  TP-0.042B  [TP-0.042B]
TP7  TP-0.042B  [TP-0.042B]
TP8  TP-0.042B  [TP-0.042B]
TP9  TP-0.042B  [TP-0.042B]
TP10  TP-1MM  [TP-0.042C]
TP11  TP-1MM  [TP-0.042C]
TP12  TP-1MM  [TP-0.042C]
U30  MIC803-40D4VM3  POR-SOT23  [SOT23]
U31  PIC32MZ1024EFE100-I/PF  MCU,PIC32MZ,TQFP-100-TQFP100_14MM  [TQFP100]
U32  LAN8720A  LOGIC,ETHERNET,LAN8720-QFN24(BIG_HOLE)  [QFN24(ONE_BIG_HOLE)]
VCO_TUNE  TP-1MM  [TP-0.042C]

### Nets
24MHZ: U31.49(OSC1/CLKI/RC12) ; also sheet 2,3
50MHZ_MAC: R93.1 U31.16(EBIA2/AN11/C2INC/ERXCLK/EREFCLK/AERX/AEREFCLK/RPG9/PMA2/RG9)
!BW_CTRL: U31.82(!SQICS1!/RPD5/RD5) ; also sheet 1
!CLK_CAL: U31.81(!SQICS0!/RPD4/RD4) ; also sheet 2
!OUT_RANGE: U31.10(AN14/C1IND/ECOL/RPG6/SCK2/RG6) ; also sheet 2
!PHY_RST: U31.17(TMS/EBIA16/AN24/RA0) U32.15(!RST)
!RIN_CTRL: U31.68(EBIA15/RPD9/PMCS2/PMA15/RD9) ; also sheet 1
!VCO_TUNE: U31.69(RPD10/SCK4/RD10) VCO_TUNE.TP ; also sheet 2
+3.3V [Power]: C123.1 C126.1 C128.1 C129.1 C130.1 C131.1 C132.1 C133.1 C134.1 C137.2 C138.1 C144.1 C145.1 L8.1(A) L9.2(B) P1.2 P2.4(TDCT) P2.5(RDCT) R85.2 R86.2 R104.1 R105.1 R107.1 R108.1 R109.1 R111.1 R112.1 SW1.C(COM) SW1.D(SW1) SW2.SW2(B) SW3.SW2(B) SW4.SW2(B) U30.3(VMON) U31.14(VDD) U31.37(VDD) U31.46(VDD) U31.52(VBUS3V3) U31.62(VDD) U31.74(VDD) U31.83(VDD) U31.93(VDD) U32.9(VDDIO) ; also sheet 1,2,3
+5USB: D3.1(V+) J8.1(VBUS) R97.2
+5VA [Power]: C120.1 DIS1.VDD ; also sheet 1
A0: U31.44(EBIA0/AN10/ERXD3/AETXD2/RPB15/OCFB/PMA0/RB15) ; also sheet 3
A1: U31.43(EBIA1/AN9/ERXD2/AETXD3/RPB14/SCK3/PMA1/RB14) ; also sheet 3
A4: U31.11(EBIA4/AN13/C1INC/ECRS/RPG7/SDA4/PMA4/RG7) ; also sheet 3
A5: U31.2(EBIA5/AN34/PMA5/RA5) ; also sheet 3
A6: U31.6(EBIA6/AN22/RPC1/PMA6/RC1) ; also sheet 3
ADC_OB/!2C: U31.96(TRD1/SQID1/RG12) ; also sheet 1
ADC_PD/!FD: U31.97(TRD0/SQID0/RG13) ; also sheet 1
AGND: C120.2 C121.1 C122.1 C123.2 C124.1 C125.1 C126.2 C127.1 C128.2 C129.2 C130.2 C131.2 C132.2 C133.2 C134.2 C135.2 C136.1 C137.1 C138.2 C139.2 C140.2 C141.2 C142.2 C143.2 C144.2 C145.2 D3.4(V-) DIS1.COM J8.4(GND) J8.S1(SHIELD) P1.3 P2.8(SHLD) P2.SHLD1(SHLD) P2.SHLD2(SHLD) R87.2 R88.2 R89.2 R90.2 R91.2 R94.2 R95.2 R96.2 R100.2 R110.1 R113.1 SW2.MTG1(CASE) SW2.MTG2(CASE) SW3.MTG1(CASE) SW3.MTG2(CASE) SW4.MTG1(CASE) SW4.MTG2(CASE) U30.1(COM) U31.13(VSS) U31.31(AVSS) U31.36(VSS) U31.45(VSS) U31.53(VSS) U31.63(VSS) U31.75(VSS) U31.84(VSS) U31.92(VSS) U32.PAD(COM) U32.PAD-DRILL(COM) ; also sheet 1,2,3
D0: U31.91(EBID0/PMD0/RE0) ; also sheet 3
D1: U31.94(EBID1/PMD1/RE1) ; also sheet 3
D2: U31.98(EBID2/PMD2/RE2) ; also sheet 3
D3: U31.99(EBID3/RPE3/PMD3/RE3) ; also sheet 3
D4: U31.100(EBID4/AN18/PMD4/RE4) ; also sheet 3
D5: U31.3(EBID5/AN17/RPE5/PMD5/RE5) ; also sheet 3
D6: U31.4(EBID6/AN16/PMD6/RE6) ; also sheet 3
D7: U31.5(EBID7/AN15/PMD7/RE7) ; also sheet 3
D8: U31.88(EBID8/RPG0/PMD8/RG0) ; also sheet 3
D9: U31.87(EBID9/ETXERR/RPG1/PMD9/RG1) ; also sheet 3
D10: U31.86(EBID10/ETXD0/RPF1/PMD10/RF1) ; also sheet 3
D11: U31.85(EBID11/ETXD1/RPF0/PMD11/RF0) ; also sheet 3
D12: U31.79(EBID12/ETXD2/RPD12/PMD12/RD12) ; also sheet 3
D13: U31.80(EBID13/ETXD3/PMD13/RD13) ; also sheet 3
D14: U31.77(EBID14/ETXEN/RPD2/PMD14/RD2) ; also sheet 3
D15: U31.78(EBID15/ETXCLK/RPD3/PMD15/RD3) ; also sheet 3
DAC_SLEEP: U31.95(TRD2/SQID2/RG14) ; also sheet 2
N$13: DIS1.RXD U31.72(SOSCI/RPC13/RC13)
N$31: C136.2 L8.2(B) U31.30(AVDD)
N$40: R96.1 SW4.SW1(A) U31.35(AN6/ERXERR/AETXERR/RB11)
N$95: R90.1 SW1.B U31.27(PGED2/AN47/RPB7/RB7)
N$102: R86.1 TP4.TP
N$107: R91.1 SW1.E(SW2) U31.33(EBIA7/AN49/RPB9/PMA7/RB9)
N$111: R85.1 TP3.TP
N$112: C122.2 TP8.TP U31.22(AN3/C2INA/RPB3/RB3)
N$113: C121.2 TP7.TP U31.23(AN2/C2INB/RPB2/RB2)
N$114: P1.5 U31.24(PGEC1/AN1/RPB1/RB1)
N$115: P1.4 U31.25(PGED1/AN0/RPB0/RB0)
N$116: C124.2 TP9.TP U31.21(AN4/C1INB/RB4)
N$117: U31.18(AN25/AERXD0/RPE8/RE8) U32.8(RXD0)
N$118: U31.19(AN26/AERXD1/RPE9/RE9) U32.7(RXD1)
N$119: U31.1(AN23/AERXERR/RG15) U32.10(RXER)
N$120: U31.47(AN32/AETXD0/RPD14/RD14) U32.17(TXD0)
N$121: U31.48(AN33/AETXD1/RPD15/SCK6/RD15) U32.18(TXD1)
N$122: U31.67(AETXEN/RPA15/SDA1/RA15) U32.16(TXEN)
N$124: U31.70(EMDC/AEMDC/RPD11/RD11) U32.13(MDC)
N$125: R105.2 U31.71(EMDIO/AEMDIO/RPD0/RTCC/INT0/RD0) U32.12(MDIO)
N$126: U31.12(EBIA3/AN12/C2IND/ERXDV/ECRSDV/AERXDV/AECRSDV/RPG8/SCL4/PMA3/RG8) U32.11(CRS_DV)
N$128: C142.1 C143.1 U32.6(VDDCR)
N$129: R110.2 U32.24(RBIAS)
N$130: P2.1(TD+) R111.2 U32.21(TXP)
N$131: P2.2(TD-) R109.2 U32.20(TXN)
N$132: P2.3(RD+) R108.2 U32.23(RXP)
N$133: P2.6(RD-) R107.2 U32.22(RXN)
N$134: C139.1 C140.1 C141.1 L9.1(A) U32.1(VDDA) U32.19(VDDA)
N$135: R104.2 U32.14(!INT)
N$136: C127.2 R98.1 U31.55(D+)
N$137: C125.2 R99.1 U31.54(D-)
N$138: P2.12(LED-RA) U32.3(LED1)
N$139: P2.10(LED-LC) U32.2(LED2)
N$141: P2.11(LED-RC) R113.2
N$142: C135.1 R97.1 U31.51(VBUS)
N$143: P2.9(LED-LA) R112.2
N$145: D3.5(B) J8.2(D-) R99.2
N$146: D3.3(A) J8.3(D+) R98.2
N$148: 50MHZ.TP R92.2 R93.2 U31.66(AETXCLK/RPA14/SCL1/RA14)
N$149: R87.1 TP5.TP
N$150: R88.1 TP6.TP
N$193: R89.1 SW1.A U31.26(PGEC2/AN46/RPB6/RB6)
N$195: R94.1 SW2.SW1(A) U31.65(EBIA8/RPF5/SCL5/PMA8/RF5)
N$196: R95.1 SW3.SW1(A) U31.32(EBIA10/AN48/RPB8/PMA10/RB8)
N$197: P1.1 U30.2(Q) U31.15(!MCLR)
N$215: R100.1 U31.73(SOSCO/RPC14/T1CK/RC14)
N$220: TP12.TP U31.64(EBIA9/RPF4/SDA5/PMA9/RF4)
N$221: TP11.TP U31.56(RPF3/USBID/RF3)
N$222: TP10.TP U31.57(EBIRDY3/RPF2/SDA3/RF2)
PGA-A0: U31.38(TCK/EBIA19/AN29/RA1) ; also sheet 1
PGA-A1: U31.59(!EBICS0!/SCL2/RA2) ; also sheet 1
PHY_50MHZ: R92.1 U32.5(CLKIN)
RD: U31.9(EBIOE/AN19/RPC4/PMRD/RC4) ; also sheet 3
RF_EXT/!INT: U31.60(EBIRDY1/SDA2/RA3) ; also sheet 2
SLO_CLK: S-CLK.TP U31.76(RPD1/SCK1/RD1) ; also sheet 1,2
SLO_DAT: S-DAT.TP U31.20(AN45/C1INA/RPB5/RB5) ; also sheet 1,2
TTL1_O/!I!: U31.61(EBIA14/PMCS1/PMA14/RA4) ; also sheet 3
TTL2_O/!I!: U31.89(TRCLK/SQICLK/RA6) ; also sheet 3
WR: U31.8(EBIWE/AN20/RPC3/PMWR/RC3) ; also sheet 3
Unconnected: U31.7(EBIA12/AN21/RPC2/PMA12/RC2) U31.28(VREF-/CVREF-/AN27/AERXD2/RA9) U31.29(VREF+/CVREF+/AN28/AERXD3/RA10) U31.34(EBIA13/CVREFOUT/AN5/RPB10/PMA13/RB10) U31.39(TDI/EBIA18/AN30/RPF13/SCK5/RF13) U31.40(TDO/EBIA17/AN31/RPF12/RF12) U31.41(EBIA11/AN7/ERXD0/AECRS/PMA11/RB12) U31.42(AN8/ERXD1/AECOL/RB13) U31.50(OSC2/CLKO/RC15) U31.58(EBIRDY2/RPF8/SCL3/RF8) U31.90(TRD3/SQID3/RA7) U32.4(XTAL2)

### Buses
D[0..15],A[0..6],RD,WR

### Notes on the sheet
- MCU-FPGA Bus
- ISP PicKit
- Pots or
- thermistors
- (ISR1)
- Quadrature
- (ISR2)
- (ISR3)
- (ISR4)
- (OC2)
- (OC1)
- (OC3)
- (G)
- (R)
- OC (PWM) for
  RGB display
  NHD-0216K3Z-NS(RGB)-FBW-V3
- (B)

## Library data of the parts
15V+ 15V- 24MHZ 50MHZ COM CONF_DONE S-CLK S-DAT TP1-TP12 VCO_TUNE = QuantumOptics:TP: Testpoint, single pin or single socket, either SMT pad, small hole or loop style TP such as Keystone 5002K (0.042").
C1 C9 C11 C13 C18 C20 = QuantumOptics:CAP-POL-: Capacitor, Polarized, SMT 0805 and up, probably tantalum.; PN: TR3D107K016C0075
C2-C8 C10 C12 C14-C16 C19 C21-C29 C31-C33 C35-C47 C49 C54-C57 C60-C68 C70 C72 C77 C79-C84 C86-C89 C120 C123 C134 C135 C137-C145 = QuantumOptics:CAP-H-: Cap, SMT and Through-hole, 0402 and up.
C17 C30 C34 C48 C50-C53 C58 C59 C69 C71 C75 C78 C85 C90-C119 C121 C122 C124-C133 C136 = QuantumOptics:CAP-V-: Cap, SMT and Through-hole, 0402 and up.
C73 C74 = QuantumOptics:CAP-H-: Cap, SMT and Through-hole, 0402 and up.; PN: 08053C225KAT2A
C76 = QuantumOptics:CAP-X2Y_DUAL: X2Y dual cap in 1608 (old 0603), for bypassing bipolar parts. Based on http://www.yageo.com/pdf/X2Y_series_12.pdf.; PN: CX0805MRX7R7BB104
D1 D2 = QuantumOptics:TVS,BIPOLAR: Biploar TVS such as ComChip ATV02W___-HF.
D3 = QuantumOptics:DIODES,ESD-PROTECTION: ESD protection diodes such as TI TPD2E001.
DIS1 = QuantumOptics:DISPLAY:3WIRE: LCD display module, serial (RS232, I2C or SPI), actually just the connector. e.g. Newhaven Display Intl NHD-0216B3Z-FL-GBW http://www.newhavendisplay.com/pdf/nhd-0216b3z-fl-gbw.pdf; MFG: Newhaven Display Intl.
F1 = QuantumOptics:FUSE: Fuse; HOLDER1: 01110005MR; HOLDER2: 01110005MR
J1-J3 = QuantumOptics:CONN:BNC,DUAL: Dual BNC, panel mount RA throughhole, Amphenol 31-657, Cinch VBI501, Bomar 364A2595 etc have shields connected, not sure about others.
J4 = QuantumOptics:CONN:BNC: BNC PCB, horizontal or vertical, e.g. Horiz: Amp (5)227677-1, nut 1-329631-2, shoulder washer 330620, vert isolated 5227222-6, http://catalog.tycoelectronics.com/TE/bin/TE.Connect?C=1&M=BYPN&TCPN=5227222-6&RQPN=5227222-6 ...
J5 J6 = QuantumOptics:CONN:BNC,DUAL: Dual BNC, panel mount RA throughhole, Amphenol 31-657, Cinch VBI501, Bomar 364A2595 etc have shields connected, not sure about others.; MFG: Bomar
J7 = QuantumOptics:CONN:2X5-BLASTER: Connector, 2x5 for xBlaster, on 0.1" grid, for Altera FPGA programmer/JTAG connectors. Can use Omron XG4C-1031.
J8 = QuantumOptics:CONN,USB-AUY1007: USB Device side Connector, Assman [sic], PCB. Square USB-B type connector for load side.
L1-L9 = QuantumOptics:INDUCTOR: Inductor, generic inductor.
P1 = QuantumOptics:CONN:1X5-TYPE1: Connector, 5-pin
P2 = QuantumOptics:CONN,RJ45_WITH_MAGNETICS_LEDS#1: RJ-45 with built-in magnetics and LEDs, such as Pulse J00-0014NL45NL/61NL/65NL.
PWR1 = QuantumOptics:DC-DC:CCP-__-E(TDK1.5-25W): CCp-inoutsc-E, TDK DC-DC isolated, 1.5-25W, uni- or bipolar "p": 1.5, 3, 6, 10, 15, or 25W. "in": Input 05, 12, 24 or 48V. "out": Output 3.3, 5, 12, ±12 (or 24), ±15 (or30V). "s": Polarity single or dual. "c": Case horiz DIP, horiz SMD or vertical SIP. http://www.tdk.co.jp/tefe02/ea335_cc_e.pdf
Q1 = QuantumOptics:MOSFET-N: Mosfet, N-Channel, generic enhancement mode N-FET, such as 2N7002 in SOT-23.
R1 R2 R4 R5 R7 R8 R11-R15 R18-R23 R26 R29-R32 R34 R36 R37 R39 R43 R44 R46 R51 R61 R65 R69 R70 R73 R76 R78 R89-R100 R104 R105 R107-R109 R111 R112 = QuantumOptics:R-H-*: Resistor, SMT & Through-Hole, horizontal symbol
R3 R6 R9 R10 R24 R25 R27 R28 R33 R38 R40-R42 R45 R47-R50 R52-R60 R62-R64 R66-R68 R71 R72 R74 R75 R77 R79-R83 R85-R88 R110 R113 = QuantumOptics:R-V-*: Resistor, SMT & Through-Hole, vertical symbol
R16 R17 R84 = QuantumOptics:R-4PAK: Quad Resistor Pack
R35 = QuantumOptics:POT: Pot, regular or trimpot; PN: 3361P-1-101G
RF1 = QuantumOptics:RF-SHIELD: RF Shield, 27 x 27 x 5mm, Laird Tech BMI-S-203-F, SMT; COVER: BMI-S-205-C
RF2 = QuantumOptics:RF-SHIELD: RF Shield, 27 x 27 x 5mm, Laird Tech BMI-S-203-F, SMT; COVER: BMI-S-207-C
RF3 = QuantumOptics:RF-SHIELD: RF Shield, 27 x 27 x 5mm, Laird Tech BMI-S-203-F, SMT; COVER: cover???
SW1 = QuantumOptics:SWITCH,QUADRATURE+PUSHSWITCH: Quadrature rotary switch with push switch such as Bourns PEC16-2220F-S0024
SW2-SW4 = QuantumOptics:SWITCH,SPST_W-CASE: Plain old SPST pushbutton, with case connections, such as AB11AH series.
TR1 = QuantumOptics:TRANSFORMER,5WIRE: Transformer, primary with centre tapped secondary
U1-U3 = QuantumOptics:REGULATOR:3PIN: LM1086-xxx, National Semiconductor, LDO, adjustable or fixed. http://cache.national.com/ds/LM/LM1086.pdf
U4 U7 = QuantumOptics:SWITCH,8PST-SERIAL: Analog switch, 8PST, serial, such as ADG1414.
U5 = QuantumOptics:ANALOG,INT-AMP-PROG#1: Instrumentation Amplifier, programmable gain, such as AD8253.
U6 U8 = QuantumOptics:OPAMP:AD8___(DUAL): AD8xxx, Analog Devices, dual opamp in SOIC-8 and MSOP-8, various versions available. AD8066, AD8656, etc. e.g. http://www.analog.com/UploadedFiles/Data_Sheets/476080131AD8655_6_a.pdf
U9 = QuantumOptics:ADC,LTC2389-16: LTC2389-16 ADC, 16-bit 2.5MSPS parallel/serial, wide input range. EP on QFN pkg only.
U10 U11 U15 = QuantumOptics:DAC,SERIAL,FDBK: DAC with output feedback, serial, ref pin, such as Analog Devices AD5620/40/60 with int ref, 3-5V, slow.
U12 = QuantumOptics:DAC,AD97X4(14-BIT,125MSPS,PAR): AD9754/64, DAC 14-bit, 125MSPS, Analog Devices, pin compaitble with 12-bit to 8-bit versions.
U13 U17 = QuantumOptics:OPAMP: Op Amp, generic, pick the right package. e.g. AD8605: SOT-23-5, RRIO, 10MHz, Ib = 1pA, Vio < 65uV, 2.7-5.5V.
U14 = QuantumOptics:OSCILLATOR:CX750(CITIZEN): CSX750 Oscillators, Citizen, +3.3V or +5V, 1MHZ to 133MHz. http://www.citizencrystal.com/images/pdf/os-csx750f.pdf
U16 = QuantumOptics:COMPARATOR,SINGLE,SINGLE_SUPPY: Comparator, single, with single supply, can be totem pole or OC, such as LM397.
U18 U24 = QuantumOptics:SWITCH,SP3T,PAR: Switch, analog, 1 of 3 (SP3T), parallel, such as HMC245AQS16E.
U19 = QuantumOptics:LINEAR,VGA,#2: VCA82x, Variable Gain Amp, T.I., various dB/V and V/V. e.g. VCA822, VCA824. Example http://focus.ti.com/docs/prod/folders/print/vca822.html
U20 = QuantumOptics:COMPARATOR,ADCMP551(DUAL,500PS,LVPECL): Comparator, ADCMP551, dual PECL 500pS
U21 = QuantumOptics:RF,AMP#1: RF Amplifier, hybrid Darlington, such as Minicircuits ERA-6(SM).
U22 = QuantumOptics:REGULATOR:NEG-3-TERM: Negative 3-Pin, such as LM2990, http://www.national.com/ds/LM/LM2990.pdf
U23 = QuantumOptics:RF,DIVIDE_BY_N: RF frequency divide by 2 or 4, such as HMC361 /2 or 362 /4, DC-10GHz +5V.; DIV: 2
U25-U28 = QuantumOptics:LOGIC,BUFFER,BIDIR,1-BIT: Buffer, Bidirectional, 1-bit such as SN74LVC1T45DBVR.
U29 = QuantumOptics:FPGA_EP4C_T144(CYCLONE4): Altera FPGA in EQFP-144 such as EP4CE Cyclone IV or MAX10.; FAMILY: MAX 10
U30 = QuantumOptics:POR: Power On Reset, either active high or low (add invert symbol). e.g. Maxim MCP809/810, http://ww1.microchip.com/downloads/en/DeviceDoc/11194c.pdf
U31 = QuantumOptics:MCU,PIC32MZ,TQFP-100: Microchip PIC32MZ, 32-bit MCU with e'net, USB, FPU, 100-pin pinout such as PIC32MZ1024EFE100-I/PF.
U32 = QuantumOptics:LOGIC,ETHERNET,LAN8720: Microchip LAN8720, ethernet phy, 10/100, RMII interface and auto-MDIX.
VCO1 = QuantumOptics:RF,VCO#1: VCO, with tunng, such as Minicircuits POS-150 or JTOS-100; PIN1: H8505; PIN2: H8505; PIN3: H8505; PIN4: H8505; PIN5: H8505; PIN6: H8505; PIN7: H8505; PIN8: H8505; SPACER1: 9913-062; SPACER2: 9913-062; SPACER3: 9913-062; SPACER4: 9913-062

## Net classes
0 default: width 0.127 mm, drill 0.203 mm, clearance 0.127 mm
1 Power: width 0.25 mm, drill 0.711 mm, clearance 0.127 mm
2 Microstrip_50: width 0.356 mm, clearance 0.508 mm
3 Power,0.25mm: width 0.25 mm, drill 0.711 mm, clearance 0.127 mm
